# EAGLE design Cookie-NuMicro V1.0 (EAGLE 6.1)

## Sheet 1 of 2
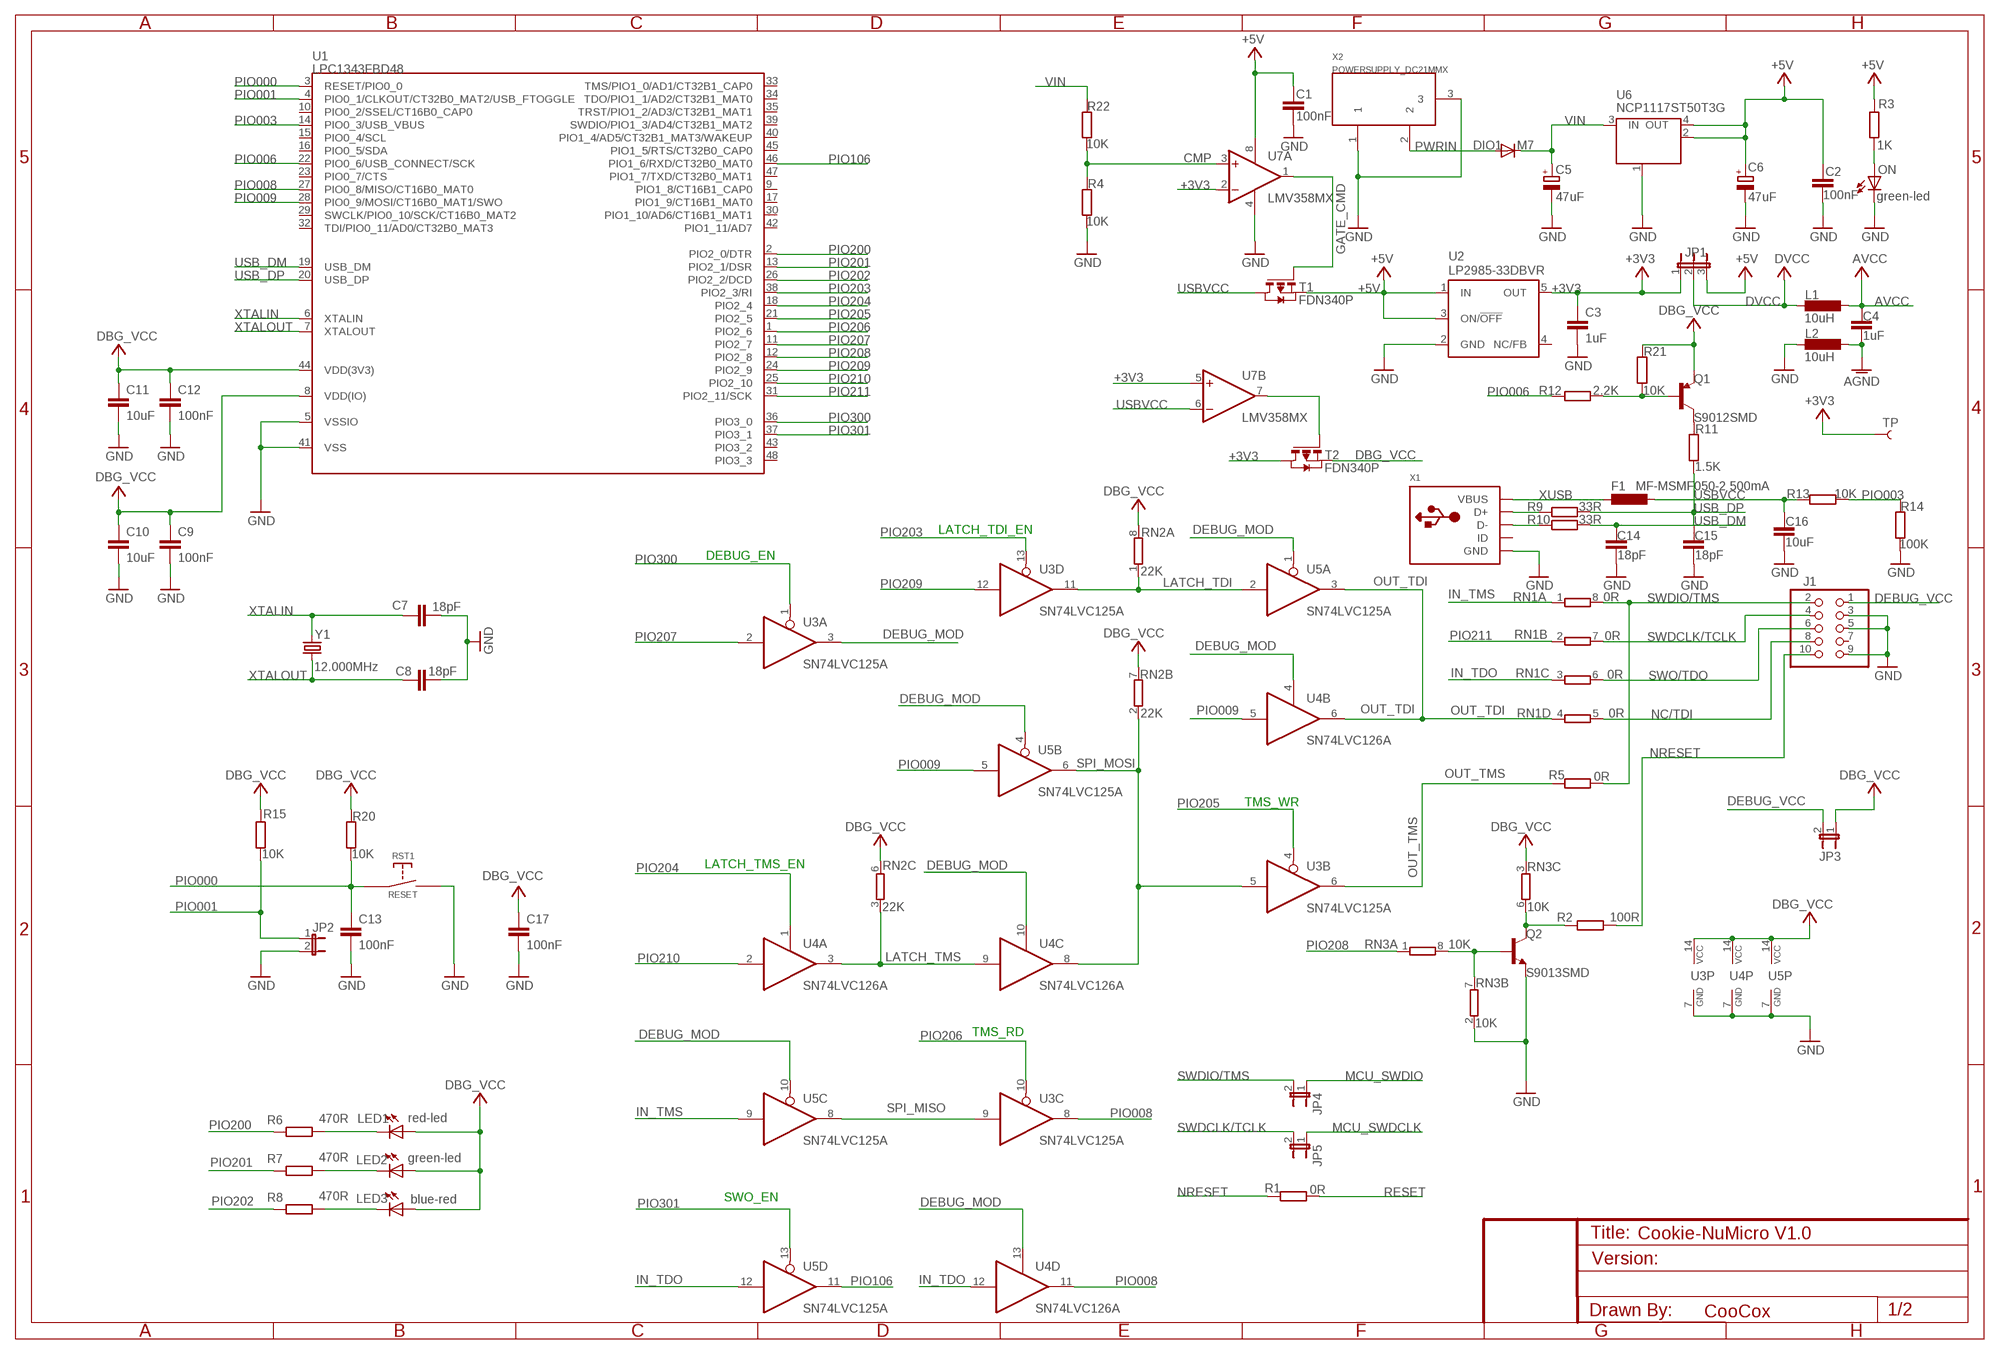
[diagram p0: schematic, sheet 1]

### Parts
C1  100nF  C-EUC0603  [C0603]
C2  100nF  C-EUC0603  [C0603]
C3  1uF  C-EUC0603  [C0603]
C4  1uF  C-EUC0603  [C0603@1]
C5  47uF  CPOL-EUD  [PANASONIC_D]
C6  47uF  CPOL-EUD  [PANASONIC_D]
C7  18pF  C-EUC0603  [C0603@1]
C8  18pF  C-EUC0603  [C0603@1]
C9  100nF  C-EUC0603  [C0603@1]
C10  10uF  C-EUC0805  [C0805]
C11  10uF  C-EUC0805  [C0805]
C12  100nF  C-EUC0603  [C0603@1]
C13  100nF  C-EUC0603  [C0603@1]
C14  18pF  C-EUC0603  [C0603@1]
C15  18pF  C-EUC0603  [C0603]
C16  10uF  C-EUC0805  [C0805]
C17  100nF  C-EUC0603  [C0603@1]
DIO1  M7  DIODE-SMB  [SMB]
F1  MF-MSMF050-2 500mA  L-EUL1812  [L1812]
J1  PINHD-2X5  [2X05]
JP1  JP2E  [JP2]
JP2  JP1E  [JP1]
JP3  JP1E  [JP1]
JP4  JP1E  [JP1]
JP5  JP1E  [JP1]
L1  10uH  L-EUL3216C  [L3216C]
L2  10uH  L-EUL3216C  [L3216C]
LED1  red-led  LEDCHIP-LED0805  [CHIP-LED0805]
LED2  green-led  LEDCHIP-LED0805  [CHIP-LED0805]
LED3  blue-red  LEDCHIP-LED0805  [CHIP-LED0805]
ON  green-led  LEDCHIP-LED0805  [CHIP-LED0805]
Q1  S9012SMD  TRANSISTOR_PNPSMD  [SOT23-3]
Q2  S9013SMD  TRANSISTOR_NPNSOT23  [SOT23]
R1  0R  R-EU_R0603  [R0603]
R2  100R  R-EU_R0603  [R0603]
R3  1K  R-EU_R0603  [R0603]
R4  10K  R-EU_R0603  [R0603]
R5  0R  R-EU_R0603  [R0603]
R6  470R  R-EU_R0603  [R0603]
R7  470R  R-EU_R0603  [R0603]
R8  470R  R-EU_R0603  [R0603]
R9  33R  R-EU_R0603  [R0603]
R10  33R  R-EU_R0603  [R0603]
R11  1.5K  R-EU_R0603  [R0603]
R12  2.2K  R-EU_R0603  [R0603]
R13  10K  R-EU_R0603  [R0603]
R14  100K  R-EU_R0603  [R0603]
R15  10K  R-EU_R0603  [R0603]
R20  10K  R-EU_R0603  [R0603]
R21  10K  R-EU_R0603  [R0603]
R22  10K  R-EU_R0603  [R0603]
RN1  0R  4R-N0603-ARV  [0603-ARV]
RN2  22K  4R-N0603-ARV  [0603-ARV]
RN3  10K  4R-N0603-ARV  [0603-ARV]
RST1  RESET  SWITCH  [TACTILE-SWITCH-1101NE]
T1  FDN340P  PMOSSOT23  [SOT-23]
T2  FDN340P  PMOSSOT23  [SOT-23]
TP  TEST-POINT3X5  [PAD.03X.05]
U1  LPC1343FBD48  [LQFP48-7X7]
U2  LP2985-33DBVR  LP2985-XXDBVR33  [SOT23-DBV]
U3  SN74LVC125A  74LVC125A  [TSSOP14]
U4  SN74LVC126A  74LVC126A  [TSSOP14]
U5  SN74LVC125A  74LVC125A  [TSSOP14]
U6  NCP1117ST50T3G  MC33269ST-3.3T3  [SOT223]
U7  LMV358MX  [SO08]
X1  USBMINIB  [USB-MINIB]
X2  POWERSUPPLY_DC21MMX  [POWERSUPPLY_DC-21MM]
Y1  12.000MHz  MC-405  [MC-405]

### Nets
+3V3: C3.1 JP1.1 T2.1(D) TP.P$1 U2.5(OUT) U7.2(A:-IN) U7.5(B:+IN) ; also sheet 2
+5V [usbvcc]: C1.1 C2.1 C6.+ JP1.3 R3.1 T1.2(S) U2.1(IN) U2.3(ON/!OFF) U6.2(OUT) U6.4(OUT) U7.8(P:V+) ; also sheet 2
AGND: C4.2 L2.2 ; also sheet 2
AVCC: C4.1 L1.2 ; also sheet 2
CMP: R4.2 R22.1 U7.3(A:+IN)
DBG_VCC [gnd]: C9.1 C10.1 C11.1 C12.1 C17.1 JP3.1 LED1.A LED2.A LED3.A Q1.2(E) R15.1 R20.2 R21.2 RN2.6 RN2.7 RN2.8 RN3.3 T2.2(S) U1.8(VDD(IO)) U1.44(VDD(3V3)) U3.14(P:VCC) U4.14(P:VCC) U5.14(P:VCC)
DEBUG_MOD: U3.3(A:O) U4.4(B:OE) U4.10(C:OE) U4.13(D:OE) U5.1(A:OE) U5.4(B:OE) U5.10(C:OE)
DEBUG_VCC: J1.1 JP3.2
DVCC: JP1.2 L1.1 ; also sheet 2
GATE_CMD: T1.3(G) U7.1(A:OUT)
GND [gnd]: C1.2 C2.2 C3.2 C5.- C6.- C7.1 C8.2 C9.2 C10.2 C11.2 C12.2 C13.2 C14.1 C15.1 C16.1 C17.2 J1.3 J1.5 J1.9 JP2.2 L2.1 ON.C Q2.2(E) R4.1 R14.1 RN3.2 RST1.P$2 U1.5(VSSIO) U1.41(VSS) U2.2(GND) U3.7(P:GND) U4.7(P:GND) U5.7(P:GND) U6.1(GND/ADJ) U7.4(P:V-) X1.GND X2.1 X2.3 ; also sheet 2
IN_TDO: RN1.3 U4.12(D:I) U5.12(D:I)
IN_TMS: RN1.1 U5.9(C:I)
LATCH_TDI: RN2.1 U3.11(D:O) U5.2(A:I)
LATCH_TMS: RN2.3 U4.3(A:O) U4.9(C:I)
MCU_SWDCLK: JP5.1 ; also sheet 2
MCU_SWDIO: JP4.1 ; also sheet 2
N$1: ON.A R3.2
N$7: T2.3(G) U7.7(B:OUT)
N$13: R9.2 X1.D+
N$14: Q1.3(C) R11.2
N$15: R10.2 X1.D-
N$16: Q1.1(B) R12.2 R21.1
N$17: LED3.C R8.2
N$19: LED2.C R7.2
N$32: LED1.C R6.2
N$33: Q2.3(C) R2.1 RN3.6
N$41: Q2.1(B) RN3.7 RN3.8
NC/TDI: J1.8 RN1.5
NRESET: J1.10 R1.2 R2.2
OUT_TDI: RN1.4 U4.6(B:O) U5.3(A:O)
OUT_TMS: R5.2 U3.6(B:O)
PIO000: C13.1 R20.1 RST1.P$1 U1.3(RESET/PIO0_0)
PIO001: JP2.1 R15.2 U1.4(PIO0_1/CLKOUT/CT32B0_MAT2/USB_FTOGGLE)
PIO003: R13.2 R14.2 U1.14(PIO0_3/USB_VBUS)
PIO006: R12.1 U1.22(PIO0_6/USB_CONNECT/SCK)
PIO008: U1.27(PIO0_8/MISO/CT16B0_MAT0) U3.8(C:O) U4.11(D:O)
PIO009: U1.28(PIO0_9/MOSI/CT16B0_MAT1/SWO) U4.5(B:I) U5.5(B:I)
PIO106: U1.46(PIO1_6/RXD/CT32B0_MAT0) U5.11(D:O)
PIO200: R6.1 U1.2(PIO2_0/DTR)
PIO201: R7.1 U1.13(PIO2_1/DSR)
PIO202: R8.1 U1.26(PIO2_2/DCD)
PIO203: U1.38(PIO2_3/RI) U3.13(D:OE)
PIO204: U1.18(PIO2_4) U4.1(A:OE)
PIO205: U1.21(PIO2_5) U3.4(B:OE)
PIO206: U1.1(PIO2_6) U3.10(C:OE)
PIO207: U1.11(PIO2_7) U3.2(A:I)
PIO208: RN3.1 U1.12(PIO2_8)
PIO209: U1.24(PIO2_9) U3.12(D:I)
PIO210: U1.25(PIO2_10) U4.2(A:I)
PIO211: RN1.2 U1.31(PIO2_11/SCK)
PIO300: U1.36(PIO3_0) U3.1(A:OE)
PIO301: U1.37(PIO3_1) U5.13(D:OE)
PWRIN [power]: DIO1.A X2.2
RESET: R1.1 ; also sheet 2
SPI_MISO: U3.9(C:I) U5.8(C:O)
SPI_MOSI: RN2.2 U3.5(B:I) U4.8(C:O) U5.6(B:O)
SWDCLK/TCLK: J1.4 JP5.2 RN1.7
SWDIO/TMS: J1.2 JP4.2 R5.1 RN1.8
SWO/TDO: J1.6 RN1.6
USB_DM: C14.2 R10.1 U1.19(USB_DM)
USB_DP: C15.2 R9.1 R11.1 U1.20(USB_DP)
USBVCC [usbvcc]: C16.2 F1.1 R13.1 T1.1(D) U7.6(B:-IN)
VIN [power]: C5.+ DIO1.C R22.2 U6.3(IN) ; also sheet 2
XTALIN: C7.2 U1.6(XTALIN) Y1.2
XTALOUT: C8.1 U1.7(XTALOUT) Y1.1
XUSB: F1.2 X1.VBUS
Unconnected: J1.7 RN2.4 RN2.5 RN3.4 RN3.5 U1.9(PIO1_8/CT16B1_CAP0) U1.10(PIO0_2/SSEL/CT16B0_CAP0) U1.15(PIO0_4/SCL) U1.16(PIO0_5/SDA) U1.17(PIO1_9/CT16B1_MAT0) U1.23(PIO0_7/CTS) U1.29(SWCLK/PIO0_10/SCK/CT16B0_MAT2) U1.30(PIO1_10/AD6/CT16B1_MAT1) U1.32(TDI/PIO0_11/AD0/CT32B0_MAT3) U1.33(TMS/PIO1_0/AD1/CT32B1_CAP0) U1.34(TDO/PIO1_1/AD2/CT32B1_MAT0) U1.35(TRST/PIO1_2/AD3/CT32B1_MAT1) U1.39(SWDIO/PIO1_3/AD4/CT32B1_MAT2) U1.40(PIO1_4/AD5/CT32B1_MAT3/WAKEUP) U1.42(PIO1_11/AD7) U1.43(PIO3_2) U1.45(PIO1_5/RTS/CT32B0_CAP0) U1.47(PIO1_7/TXD/CT32B0_MAT1) U1.48(PIO3_3) U2.4(NC/FB) X1.ID

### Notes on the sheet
- LATCH_TDI_EN
- DEBUG_EN
- TMS_WR
- LATCH_TMS_EN
- TMS_RD
- SWO_EN
- CooCox

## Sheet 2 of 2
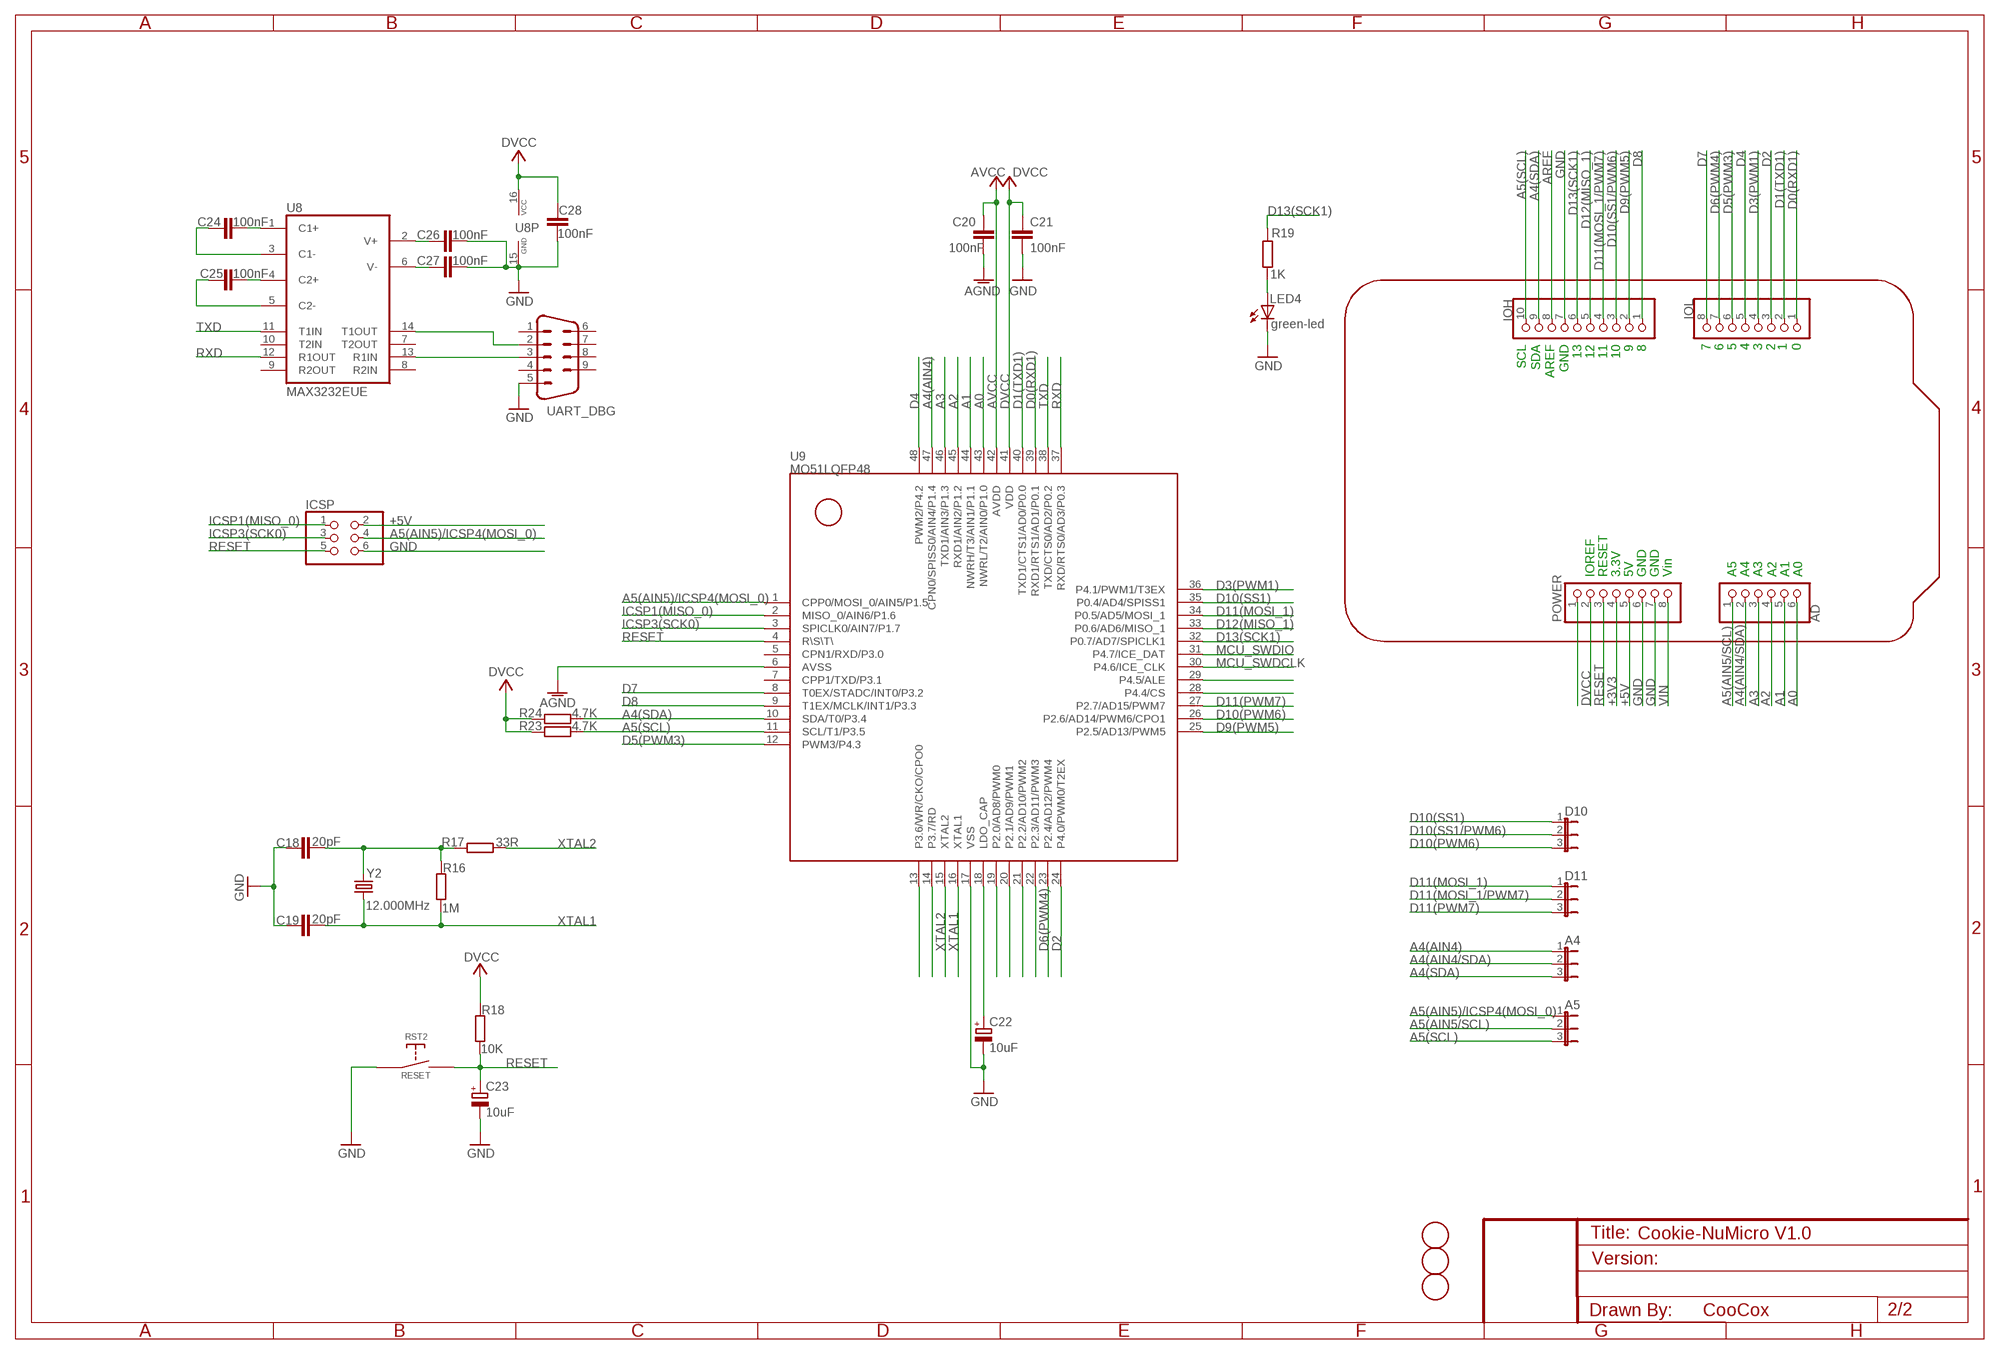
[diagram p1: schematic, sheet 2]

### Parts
A4  JP2E  [JP2]
A5  JP2E  [JP2]
AD  PINHD-1X6  [1X06]
C18  20pF  C-EUC0603  [C0603@1]
C19  20pF  C-EUC0603  [C0603@1]
C20  100nF  C-EUC0603  [C0603@1]
C21  100nF  C-EUC0603  [C0603@1]
C22  10uF  CPOL-EUSMCB  [SMC_B]
C23  10uF  CPOL-EUSMCB  [SMC_B]
C24  100nF  C-EUC0603  [C0603@1]
C25  100nF  C-EUC0603  [C0603@1]
C26  100nF  C-EUC0603  [C0603@1]
C27  100nF  C-EUC0603  [C0603@1]
C28  100nF  C-EUC0603  [C0603@1]
D10  JP2E  [JP2]
D11  JP2E  [JP2]
FD1  FIDUCIALMOUNT  [FIDUCIA-MOUNT]
FD2  FIDUCIALMOUNT  [FIDUCIA-MOUNT]
FD3  FIDUCIALMOUNT  [FIDUCIA-MOUNT]
ICSP  PINHD-2X3  [2X03]
IOH  PINHD-1X10_ARD  [1X10]
IOL  PINHD-1X8  [1X08]
LED4  green-led  LEDCHIP-LED0805  [CHIP-LED0805]
POWER  PINHD-1X8  [1X08]
R16  1M  R-EU_R0603  [R0603]
R17  33R  R-EU_R0603  [R0603]
R18  10K  R-EU_R0603  [R0603]
R19  1K  R-EU_R0603  [R0603]
R23  4.7K  R-EU_R0603  [R0603]
R24  4.7K  R-EU_R0603  [R0603]
RST2  RESET  SWITCH  [TACTILE-SWITCH-1101NE]
U8  MAX3232EUE  [TSSOP16]
U9  MO51LQFP48  [LQFP48]
UART_DBG  M09S_OBVERSE  [M09S_OBV]
Y2  12.000MHz  MC-405  [MC-405]

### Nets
+3V3: POWER.4 ; also sheet 1
+5V [usbvcc]: ICSP.2 POWER.5 ; also sheet 1
A0: AD.6 U9.43(NWRL/T2/AIN0/P1.0)
A1: AD.5 U9.44(NWRH/T3/AIN1/P1.1)
A2: AD.4 U9.45(RXD1/AIN2/P1.2)
A3: AD.3 U9.46(TXD1/AIN3/P1.3)
A4(AIN4): A4.1 U9.47(CPN0/SPISS0/AIN4/P1.4)
A4(AIN4/SDA): A4.2 AD.2
A4(SDA): A4.3 IOH.9 R24.1 U9.10(SDA/T0/P3.4)
A5(AIN5)/ICSP4(MOSI_0): A5.1 ICSP.4 U9.1(CPP0/MOSI_0/AIN5/P1.5)
A5(AIN5/SCL): A5.2 AD.1
A5(SCL): A5.3 IOH.10 R23.1 U9.11(SCL/T1/P3.5)
AGND: C20.2 U9.6(AVSS) ; also sheet 1
AREF: IOH.8
AVCC: C20.1 U9.42(AVDD) ; also sheet 1
D0(RXD1): IOL.1 U9.39(RXD1/RTS1/AD1/P0.1)
D1(TXD1): IOL.2 U9.40(TXD1/CTS1/AD0/P0.0)
D2: IOL.3 U9.24(P4.0/PWM0/T2EX)
D3(PWM1): IOL.4 U9.36(P4.1/PWM1/T3EX)
D4: IOL.5 U9.48(PWM2/P4.2)
D5(PWM3): IOL.6 U9.12(PWM3/P4.3)
D6(PWM4): IOL.7 U9.23(P2.4/AD12/PWM4)
D7: IOL.8 U9.8(T0EX/STADC/INT0/P3.2)
D8: IOH.1 U9.9(T1EX/MCLK/INT1/P3.3)
D9(PWM5): IOH.2 U9.25(P2.5/AD13/PWM5)
D10(PWM6): D10.3 U9.26(P2.6/AD14/PWM6/CPO1)
D10(SS1): D10.1 U9.35(P0.4/AD4/SPISS1)
D10(SS1/PWM6): D10.2 IOH.3
D11(MOSI_1): D11.1 U9.34(P0.5/AD5/MOSI_1)
D11(MOSI_1/PWM7): D11.2 IOH.4
D11(PWM7): D11.3 U9.27(P2.7/AD15/PWM7)
D12(MISO_1): IOH.5 U9.33(P0.6/AD6/MISO_1)
D13(SCK1): IOH.6 R19.1 U9.32(P0.7/AD7/SPICLK1)
DVCC: C21.1 C28.1 POWER.2 R18.2 R23.2 R24.2 U8.16(VCC) U9.41(VDD) ; also sheet 1
GND [gnd]: C18.1 C19.1 C21.2 C22.- C23.- C26.2 C27.2 C28.2 ICSP.6 IOH.7 LED4.C POWER.6 POWER.7 RST2.P$1 U8.15(GND) U9.17(VSS) UART_DBG.5 ; also sheet 1
ICSP1(MISO_0): ICSP.1 U9.2(MISO_0/AIN6/P1.6)
ICSP3(SCK0): ICSP.3 U9.3(SPICLK0/AIN7/P1.7)
MCU_SWDCLK: U9.30(P4.6/ICE_CLK) ; also sheet 1
MCU_SWDIO: U9.31(P4.7/ICE_DAT) ; also sheet 1
N$2: LED4.A R19.2
N$3: C24.2 U8.1(C1+)
N$4: C24.1 U8.3(C1-)
N$5: C25.2 U8.4(C2+)
N$6: C25.1 U8.5(C2-)
N$8: U8.14(T1OUT) UART_DBG.2
N$9: U9.29(P4.5/ALE)
N$10: U9.28(P4.4/CS)
N$11: C26.1 U8.2(V+)
N$12: C27.1 U8.6(V-)
N$36: POWER.1
N$38: U9.13(P3.6/WR/CKO/CPO0)
N$39: U9.14(P3.7/RD)
N$40: C18.2 R16.2 R17.2 Y2.2
N$42: U8.13(R1IN) UART_DBG.3
N$43: C22.+ U9.18(LDO_CAP)
N$44: U9.19(P2.0/AD8/PWM0)
N$45: U9.20(P2.1/AD9/PWM1)
N$46: U9.21(P2.2/AD10/PWM2)
N$47: U9.22(P2.3/AD11/PWM3)
RESET: C23.+ ICSP.5 POWER.3 R18.1 RST2.P$2 U9.4(R\S\T\) ; also sheet 1
RXD: U8.12(R1OUT) U9.37(RXD/RTS0/AD3/P0.3)
TXD: U8.11(T1IN) U9.38(TXD/CTS0/AD2/P0.2)
VIN [power]: POWER.8 ; also sheet 1
XTAL1: C19.2 R16.1 U9.16(XTAL1) Y2.1
XTAL2: R17.1 U9.15(XTAL2)
Unconnected: U8.7(T2OUT) U8.8(R2IN) U8.9(R2OUT) U8.10(T2IN) U9.5(CPN1/RXD/P3.0) U9.7(CPP1/TXD/P3.1) UART_DBG.1 UART_DBG.4 UART_DBG.6 UART_DBG.7 UART_DBG.8 UART_DBG.9

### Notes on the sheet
- SCL | SDA | AREF | GND | 13 | 12 | 11 | 10 | 9 | 8 | 7 | 6 | 5 | 4 | 3 | 2 | 1 | 0
- IOREF | RESET | 3.3V | 5V | GND | GND | Vin | A5 | A4 | A3 | A2 | A1 | A0
- CooCox

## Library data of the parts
A4 A5 D10 D11 JP1 = jumper:JP2E: JUMPER
AD = SmartPrj:PINHD-1X6: PIN HEADER
C1-C3 C15 C16 = resistor:C-EU: CAPACITOR, European symbol
C4 C7-C14 C17-C21 C24-C28 = rcl:C-EU: CAPACITOR, European symbol
C5 C6 C22 C23 = rcl:CPOL-EU: POLARIZED CAPACITOR, European symbol
DIO1 = diode:DIODE-: DIODE
F1 L1 L2 = rcl:L-EU: INDUCTOR, European symbol
FD1-FD3 = SmartPrj:FIDUCIALMOUNT
ICSP = pinhead:PINHD-2X3: PIN HEADER
IOH = SmartPrj:PINHD-1X10_ARD: PIN HEADER
IOL POWER = SmartPrj:PINHD-1X8: PIN HEADER
J1 = pinhead:PINHD-2X5: PIN HEADER
JP2-JP5 = jumper:JP1E: JUMPER
LED1-LED4 ON = led:LED: LED
Q1 = SparkFunEagle-100301:TRANSISTOR_PNP
Q2 = SparkFunEagle-100301:TRANSISTOR_NPN: Transistor NPN BJT configuration in SOT23 package. MMBT2222 is the common NPN we use. Double check BCE configuration again layout.
R1 R3-R12 R15-R24 = rcl:R-EU_: RESISTOR, European symbol
R2 R13 R14 = resistor:R-EU_: RESISTOR, European symbol
RN1-RN3 = resistor-dil:4R-N: Array Chip Resistor Source: RS Component / Phycomp; OC_FARNELL: unknown; OC_NEWARK: unknown
RST1 RST2 = SWITCH1:SWITCH
T1 T2 = zetex:PMOSSOT23: MOS FET
TP = SparkFunEagle-100301:TEST-POINT
U1 = lpc1xxx-v6:LPC1343FBD48: LPC1343 72 MHz 32-bit ARM Cortex-M3 based microcontroller featuring a high level of integration and low power consumption. 32 kB Flash, 8 kB SRAM, USB Device MarcVl - Datasheet available on www.nxp.com
U2 = SmartPrj:LP2985-XXDBVR: ULTRALOW-POWER 50-mA LOW-DROPOUT LINEAR REGULATORS 50-mA Low-Dropout Regulator Source: http://focus.ti.com/lit/ds/symlink/tps77001.pdf
U3 U5 = 74xx-eu:74*125: Quad bus BUFFER, 3-state
U4 = 74xx-eu:74*126: Quad bus BUFFER, 3-state
U6 = linear:MC33269ST*: Adjustable Output Low Dropout Voltage Regulator 800 mA Source: http://www.onsemi.com/pub/Collateral/MC33269-D.PDF
U7 = linear:LMV358?*: Dual General Purpose, Low Voltage, Rail-to-Rail Output Operational Amplifiers Source: http://www.national.com/mpf/LM/LMV321.html http://www.national.com/dt/lmv_qual.pdf
U8 = maxim:MAX3232*: True RS-232 Transceivers 3.0V to 5.5V, Low-Power up to 1Mbps, Using Four 0.1µF External Capacitors Source: http://pdfserv.maxim-ic.com/en/ds/MAX3222-MAX3241.pdf; MF: MAXIM; MPN: MAX3232EUE+; OC_FARNELL: 1379769; OC_NEWARK: 68K4632
U9 = NuMicro:MO51
UART_DBG = con-subd:M09: SUB-D
X1 = adafruit:USB: USB Connectors USBMINIB - Surface Mount Female Mini-B USB Connector 4UConnector: 06564 By microbuilder.eu Thru-hole RA Female Mini-B USB Connector 4UConnector: 18732 By ladyada.net
X2 = SmartPrj:POWERSUPPLY_DC21MM
Y1 Y2 = untitled:MC-405: kHz RANGE CRYSTAL UNIT SMD; OC_FARNELL: unknown; OC_NEWARK: unknown

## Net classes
1 power: width 0.61 mm, drill 0.61 mm, clearance 0.254 mm
2 gnd: width 0.305 mm, drill 0.559 mm, clearance 0.254 mm
3 usbvcc: width 0.508 mm, drill 0.61 mm, clearance 0.254 mm

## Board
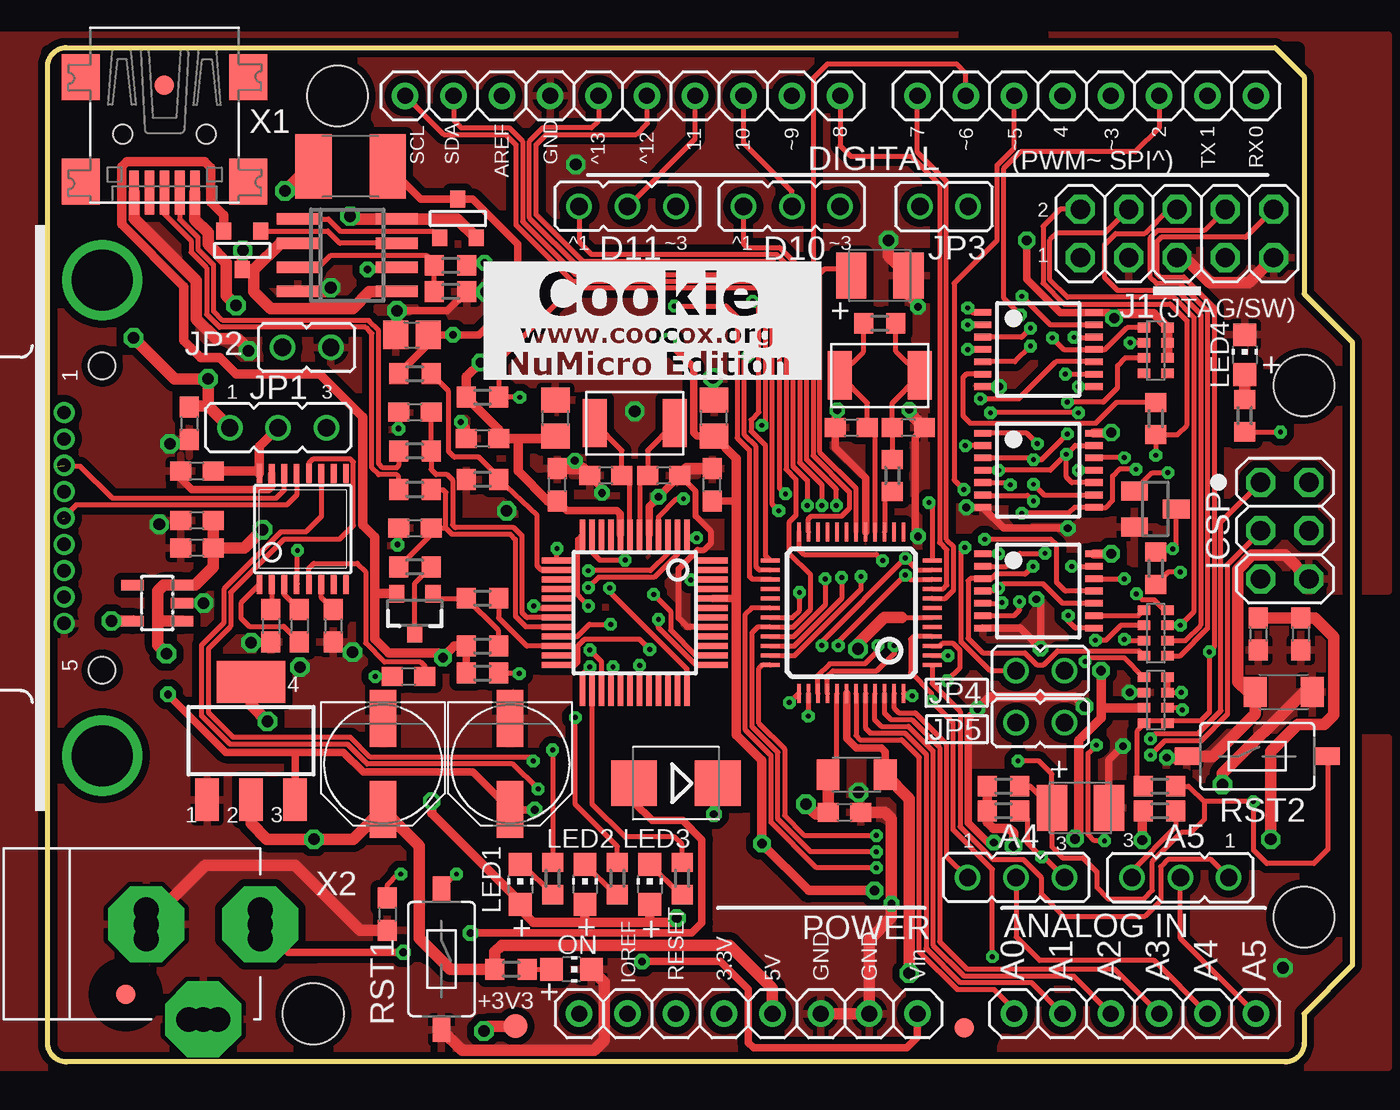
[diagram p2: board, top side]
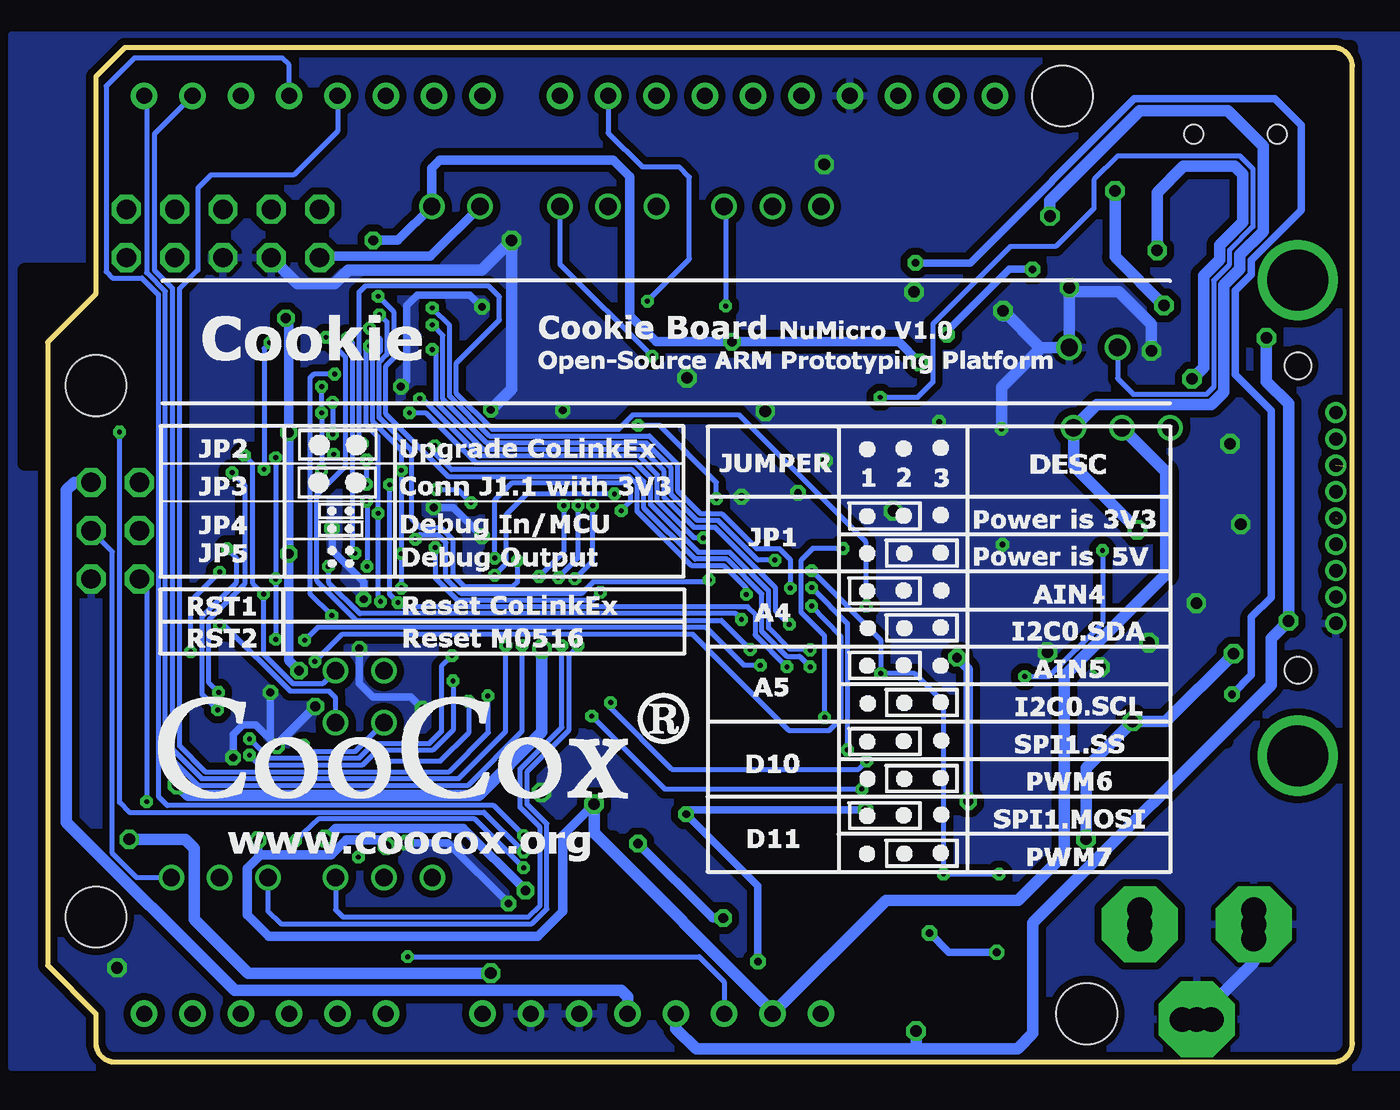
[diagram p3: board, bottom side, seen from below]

Size 68.58 x 53.34 mm. Coordinates in mm from the lower left corner, seen from the top.
Outline: 64.52,53.34 66.04,51.82 66.04,40.39 68.58,37.85 68.58,5.08 66.04,2.54 66.04,1 arc-90 65.04,0 1,0 arc-90 0,1 0,52.34 arc-90 1,53.34 64.52,53.34
Copper layers (1*16): Top 0.035mm / dielectric 1.5mm / Bottom 0.035mm
Design rules: minimum track width 6mil, minimum drill 6mil, track to track 4mil, track to pad 4mil, pad to pad 4mil, via to via 4mil, smd to smd 0mil, copper to edge 10mil, drill to drill 6mil, minimum pad ring 8mil, minimum via ring 8mil, stop-mask expansion 0mil, vias tented up to drill 100mil, thermal gap 10mil
Holes 3.2 mm at 66.04,35.56 66.04,7.62 15.24,50.8 13.97,2.54
tRestrict: area 3.1,2.5 to 5.1,4.6; area 47.2,0.8 to 49.2,2.8; area 5.1,50.3 to 7.2,52.4; area 9.7,43.9 to 10.7,44.9; area 5.3,37.9 to 6,41.4; area 4.9,38.4 to 5.3,40.5; area 4.4,38.6 to 5,39.9; area 5.9,37.3 to 6.5,40.9; area 6.2,36.6 to 7.2,37.6; area 0.3,42.4 to 3.6,45.1; area 0,46.9 to 14.9,53.1; area 14.9,45.1 to 16.8,49.2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
bRestrict: area 2.7,20.5 to 3.1,20.9; area 2.7,36.5 to 3.1,36.9; area 45.1,29.6 to 46.6,30.7; area 48.3,32.8 to 49.4,33.8; area 48.2,30.6 to 49,31.3; area 54.3,22.8 to 55.7,24.3; area 57.2,22.5 to 59.3,24.5; area 44.6,19.3 to 47.3,22.3; area 44.1,13 to 45.1,14.7; area 61.6,8 to 62.5,9.1; area 62.5,10 to 64.7,11.3; area 65.9,8.6 to 68.1,11.9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

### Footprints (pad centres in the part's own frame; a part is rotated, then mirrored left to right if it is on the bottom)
JP2 = drill 0.914 long: 1 -2.54,0; 2 0,0; 3 2.54,0
1X06 = drill 0.85 pad 1.422 long: 1 -6.35,0; 2 -3.81,0; 3 -1.27,0; 4 1.27,0; 5 3.81,0; 6 6.35,0
C0603 = smd 1.1 x 1: 1 -0.85,0; 2 0.85,0
PANASONIC_D = smd 3 x 1.4: + 2.4,0; - -2.4,0
C0805 = smd 1.3 x 1.5: 1 -0.95,0; 2 0.95,0
C0805' = smd 1.3 x 1.5: 1 -0.85,0; 2 0.85,0
SMC_B = smd 1.6 x 2.4: + -1.5,0; - 1.5,0
SMB = smd 2.4 x 2.4: A 2.2,0; C -2.2,0
L1812 = smd 1.9 x 3.4: 1 -1.95,0; 2 1.95,0
FIDUCIA-MOUNT = smd 1.016 x 1.016: P$1 0,0
2X03 = drill 1.016 octagon: 1 -2.54,-1.27; 2 -2.54,1.27; 3 0,-1.27; 4 0,1.27; 5 2.54,-1.27; 6 2.54,1.27
1X10 = drill 0.85 pad 1.422 long: 1 -11.43,0; 2 -8.89,0; 3 -6.35,0; 4 -3.81,0; 5 -1.27,0; 6 1.27,0; 7 3.81,0; 8 6.35,0; 9 8.89,0; 10 11.43,0
1X08 = drill 0.85 pad 1.422 long: 1 -8.89,0; 2 -6.35,0; 3 -3.81,0; 4 -1.27,0; 5 1.27,0; 6 3.81,0; 7 6.35,0; 8 8.89,0
2X05 = drill 1.016 octagon: 1 -5.08,-1.27; 2 -5.08,1.27; 3 -2.54,-1.27; 4 -2.54,1.27; 5 0,-1.27; 6 0,1.27; 7 2.54,-1.27; 8 2.54,1.27; 9 5.08,-1.27; 10 5.08,1.27
JP1 = drill 0.914 long: 1 0,-1.27; 2 0,1.27
L3216C = smd 1.2 x 1.6: 1 -1.5,0; 2 1.5,0
CHIP-LED0805 = smd 1.2 x 1.2: A 0,-1.05; C 0,1.05
SOT23-3 = smd 0.8 x 0.9: 1 -0.95,-1; 2 0.95,-1; 3 0,1.1
SOT23 = smd 1 x 1.4: 1 -0.95,-1.1; 2 0.95,-1.1; 3 0,1.1
R0603 = smd 1 x 1.1: 1 -0.85,0; 2 0.85,0
0603-ARV = smd 0.5 x 0.65: 1 -1.2,-0.625; 2 -0.4,-0.625; 3 0.4,-0.625; 4 1.2,-0.625; 5 1.2,0.625; 6 0.4,0.625; 7 -0.4,0.625; 8 -1.2,0.625
TACTILE-SWITCH-1101NE = smd 1.27 x 0.914: P$1 -3.708,0; P$2 3.708,0
SOT-23 = smd 0.787 x 0.889: 1 0.025,-1.016; 2 -0.94,1.016; 3 0.991,1.016
PAD.03X.05 = smd 1.27 x 1.27: P$1 0,0
LQFP48-7X7 = smd 0.3 x 1.6: 1 -2.75,-4.1; 2 -2.25,-4.1; 3 -1.75,-4.1; 4 -1.25,-4.1; 5 -0.75,-4.1; 6 -0.25,-4.1; 7 0.25,-4.1; 8 0.75,-4.1; 9 1.25,-4.1; 10 1.75,-4.1; 11 2.25,-4.1; 12 2.75,-4.1; 25 2.75,4.1; 26 2.25,4.1; 27 1.75,4.1; 28 1.25,4.1; 29 0.75,4.1; 30 0.25,4.1; 31 -0.25,4.1; 32 -0.75,4.1; 33 -1.25,4.1; 34 -1.75,4.1; 35 -2.25,4.1; 36 -2.75,4.1 | smd 1.6 x 0.3: 13 4.1,-2.75; 14 4.1,-2.25; 15 4.1,-1.75; 16 4.1,-1.25; 17 4.1,-0.75; 18 4.1,-0.25; 19 4.1,0.25; 20 4.1,0.75; 21 4.1,1.25; 22 4.1,1.75; 23 4.1,2.25; 24 4.1,2.75; 37 -4.1,2.75; 38 -4.1,2.25; 39 -4.1,1.75; 40 -4.1,1.25; 41 -4.1,0.75; 42 -4.1,0.25; 43 -4.1,-0.25; 44 -4.1,-0.75; 45 -4.1,-1.25; 46 -4.1,-1.75; 47 -4.1,-2.25; 48 -4.1,-2.75
SOT23-DBV = smd 0.55 x 1.2: 1 -0.95,-1.3; 2 0,-1.3; 3 0.95,-1.3; 4 0.95,1.3; 5 -0.95,1.3
TSSOP14 = smd 0.35 x 0.9: 1 -1.95,-2.925; 2 -1.3,-2.925; 3 -0.65,-2.925; 4 0,-2.925; 5 0.65,-2.925; 6 1.3,-2.925; 7 1.95,-2.925; 8 1.95,2.925; 9 1.3,2.925; 10 0.65,2.925; 11 0,2.925; 12 -0.65,2.925; 13 -1.3,2.925; 14 -1.95,2.925
SOT223 = smd 1.219 x 2.235: 1 -2.311,-3.099; 2 0,-3.099; 3 2.311,-3.099 | smd 3.6 x 2.2: 4 0,3.099
SO08 = smd 0.6 x 2.2: 1 -1.905,-2.6; 2 -0.635,-2.6; 3 0.635,-2.6; 4 1.905,-2.6; 5 1.905,2.6; 6 0.635,2.6; 7 -0.635,2.6; 8 -1.905,2.6
TSSOP16 = smd 0.305 x 0.991: 1 -2.275,-2.918; 2 -1.625,-2.918; 3 -0.975,-2.918; 4 -0.325,-2.918; 5 0.325,-2.918; 6 0.975,-2.918; 7 1.625,-2.918; 8 2.275,-2.918; 9 2.275,2.918; 10 1.625,2.918; 11 0.975,2.918; 12 0.325,2.918; 13 -0.325,2.918; 14 -0.975,2.918; 15 -1.625,2.918; 16 -2.275,2.918
LQFP48 = smd 0.2 x 1: 1 -2.75,-4.25; 2 -2.25,-4.25; 3 -1.75,-4.25; 4 -1.25,-4.25; 5 -0.75,-4.25; 6 -0.25,-4.25; 7 0.25,-4.25; 8 0.75,-4.25; 9 1.25,-4.25; 10 1.75,-4.25; 11 2.25,-4.25; 12 2.75,-4.25; 25 2.75,4.25; 26 2.25,4.25; 27 1.75,4.25; 28 1.25,4.25; 29 0.75,4.25; 30 0.25,4.25; 31 -0.25,4.25; 32 -0.75,4.25; 33 -1.25,4.25; 34 -1.75,4.25; 35 -2.25,4.25; 36 -2.75,4.25 | smd 1 x 0.2: 13 4.25,-2.75; 14 4.25,-2.25; 15 4.25,-1.75; 16 4.25,-1.25; 17 4.25,-0.75; 18 4.25,-0.25; 19 4.25,0.25; 20 4.25,0.75; 21 4.25,1.25; 22 4.25,1.75; 23 4.25,2.25; 24 4.25,2.75; 37 -4.25,2.75; 38 -4.25,2.25; 39 -4.25,1.75; 40 -4.25,1.25; 41 -4.25,0.75; 42 -4.25,0.25; 43 -4.25,-0.25; 44 -4.25,-0.75; 45 -4.25,-1.25; 46 -4.25,-1.75; 47 -4.25,-2.25; 48 -4.25,-2.75
M09S_OBV = drill 0.7: 1 5.34,2; 2 2.57,2; 3 -0.2,2; 4 -2.97,2; 5 -5.74,2; 6 3.955,2; 7 1.185,2; 8 -1.585,2; 9 -4.355,2 | drill 3.2: P$1 -12.7,0; P$2 12.3,0 | hole 1.4: -8.2,0; 7.8,0
USB-MINIB = smd 0.5 x 2.308: D+ 0,4.064; D- -0.8,4.064; GND 1.6,4.064; ID 0.8,4.064; VBUS -1.6,4.064 | smd 2 x 2.4: GND1 -4.4,-2; GND2 -4.4,3.5; GND3 4.4,3.5; GND4 4.4,-2 | hole 1: -2.2,1; 2.2,1
POWERSUPPLY_DC-21MM = drill 1.3 pad 4 octagon: 1 -5.08,-3.353; 2 -0.076,-6.35; 3 -0.076,-0.356 | drill 1.3: 4 -5.08,-4.115; 5 -5.08,-2.591; 6 -0.838,-0.356; 7 0.686,-0.356; 8 -0.838,-6.35; 9 0.686,-6.35
MC-405 = smd 1.27 x 2.54: 1 -2.108,0.013; 2 2.108,0.012

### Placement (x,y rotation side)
A4  50.9,9.7 0 top
A5  59.54,9.7 180 top
AD  57.15,2.54 180 top
C1  7.85,27.03 180 top
C2  7.85,28.47 180 top
C3  7.44,33.58 270 top
C4  1uF  [C0603]  63.63,22.5 270 top
C5  24.31,15.67 270 top
C6  17.63,15.67 270 top
C7  18pF  [C0603]  32.38,30.84 180 top
C8  18pF  [C0603]  29.34,30.84 180 top
C9  100nF  [C0603]  26.8,30.35 90 top
C10  26.7,33.86 90 top
C11  35.03,33.86 90 top
C12  100nF  [C0603]  34.92,30.35 90 top
C13  100nF  [C0603]  17.86,7.77 270 top
C14  18pF  [C0603]  19.3,34.16 0 top
C15  19.3,28.07 0 top
C16  10uF  [C0805']  19.15,38.23 0 top
C17  100nF  [C0603]  22.86,32.79 180 top
C18  20pF  [C0603]  45.24,33.35 180 top
C19  20pF  [C0603]  42.24,33.35 0 top
C20  100nF  [C0603]  65.86,22.5 270 top
C21  100nF  [C0603]  41.88,13.13 0 top
C22  43.74,41.35 0 top
C23  54.28,13.36 0 top
C24  100nF  [C0603]  13.23,22.94 270 top
C25  100nF  [C0603]  18.97,20.27 180 top
C26  100nF  [C0603]  11.73,22.94 270 top
C27  100nF  [C0603]  15.01,22.94 270 top
C28  100nF  [C0603]  7.85,31.06 180 top
D10  39.12,44.98 0 top
D11  30.48,44.98 0 top
DIO1  33.02,14.66 180 top
F1  15.93,47.09 180 top
FD1  48.18,1.8 0 top
FD2  6.12,51.36 0 top
FD3  4.11,3.56 0 top
ICSP  65.02,27.94 270 top
IOH  30.23,50.8 180 top
IOL  54.61,50.8 180 top
J1  59.36,43.56 0 top
JP1  12.12,33.35 0 top
JP2  13.61,37.57 270 top
JP3  47.12,44.98 90 top
JP4  52.17,20.57 270 top
JP5  52.17,17.83 270 top
L1  42.52,15.11 0 top
L2  64.97,19.46 0 top
LED1  24.84,9.35 0 top
LED2  28.24,9.35 0 top
LED3  31.65,9.35 0 top
LED4  62.92,37.19 0 top
ON  27.53,4.88 270 top
POWER  36.83,2.54 0 top
Q1  19.3,23.62 180 top
Q2  58.22,29.08 270 top
R1  58.45,14.5 180 top
R2  58.24,25.96 270 top
R3  24.36,4.88 0 top
R4  21.18,40.51 180 top
R5  58.24,33.83 90 top
R6  26.54,9.65 270 top
R7  29.95,9.65 270 top
R8  33.35,9.65 270 top
R9  19.3,30.1 180 top
R10  19.3,32.13 180 top
R11  19.3,26.04 0 top
R12  22.86,24.38 180 top
R13  19.3,36.2 0 top
R14  22.86,30.63 0 top
R15  22.86,34.95 0 top
R16  43.74,38.84 0 top
R17  44.4,30.84 90 top
R18  50.24,14.5 180 top
R19  62.92,33.99 90 top
R20  22.86,20.45 180 top
R21  22.86,21.87 180 top
R22  21.18,41.88 0 top
R23  58.45,13.21 180 top
R24  50.24,13.21 180 top
RN1  58.24,22.56 270 top
RN2  58.24,37.41 270 top
RN3  58.24,19.02 270 top
RST1  20.7,5.41 270 top
RST2  63.58,16.08 0 top
T1  21.59,44.35 180 top
T2  10.21,42.67 0 top
TP  24.59,1.88 0 top
U1  30.86,23.62 180 top
U2  5.77,24.13 90 top
U3  52.07,37.47 270 top
U4  52.07,31.12 270 top
U5  52.07,24.77 270 top
U6  10.69,16.89 0 top
U7  15.75,42.42 270 top
U8  13.41,28.02 0 top
U9  42.24,23.62 90 top
UART_DBG  2.87,28.8 90 top
X1  6.15,49.78 180 top
X2  4.83,7.32 90 top
Y1  30.86,33.58 0 top
Y2  43.74,36.09 0 top

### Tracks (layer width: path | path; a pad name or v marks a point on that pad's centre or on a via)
+3V3  (via drill 0.61)
  Top 0.61: U7.5 16.92,40.51 16.03,39.62 11.74,39.62 10.85,40.51 10.85,41.66 | U7.2 12.24,43.05 10.85,41.66 | 10.85,41.66 T2.1 10.24,42.65 v10.26,42.67 | JP1.1 8.43,34.49 | 8.43,34.49 7.68,34.49 C3.1 7.62,34.17 | v4.52,38.07 6.68,35.92 v8.43,35.92 8.43,34.49 | U2.5 4.46,23.19 v3.35,23.19 | TP.P$1 23.19,1.88 v22.94,1.63
  Bottom 0.61: v10.26,42.67 10.26,45.72 8.89,47.09 6.17,47.09 5.77,46.69 5.77,44.17 6.99,42.95 6.99,42.19 7.82,41.35 7.82,36.53 v8.43,35.92 | POWER.4 35.56,1.75 34.49,0.69 22.73,0.69 | 22.73,0.69 17.6,0.69 16.79,1.5 16.79,7.32 4.27,19.84 4.27,22.28 v3.35,23.19 3.35,34.62 4.52,35.79 v4.52,38.07 | v22.94,1.63 22.94,0.89 22.73,0.69
+5V  (via drill 0.61)
  Top 0.61: T1.2 21.54,44.32 U7.8 16.05,44.32 v15.9,44.48 | 38.1,3.43 POWER.5 38.1,3.89 35.84,6.15 23.88,6.15 23.51,5.78 R3.1 21.16,4.88 19.53,6.5 19.53,11.37 C6.+ 16.07,11.71 v14,11.71 11.53,11.71 10.69,12.55 U6.2 | C1.1 10.34,27.03 v11.3,27.99 | C1.1 C2.1 | C1.1 8.7,26.03 7.75,25.08 U2.3 6.11,25.08 5.79,24.77 5.79,23.19 | v6.25,21.46 5.79,21.92 5.79,23.19 | U2.1 7.06,23.19 5.79,23.19 | v11.56,17.91 10.69,18.77 U6.4
  Bottom 0.61: v15.9,44.48 15.9,45.29 11.18,50.01 6.55,50.01 4.7,48.16 4.7,43.66 5.92,42.44 5.92,41.68 6.76,40.84 6.76,35.23 7.42,34.57 13.44,34.57 JP1.3 14.66,31.34 v11.3,27.99 | ICSP.2 67.18,30.48 67.59,30.07 67.59,12.6 58.75,3.76 38.43,3.76 38.1,3.43 POWER.5 | v14,11.71 14,15.47 v11.56,17.91 9.8,17.91 v6.25,21.46
A0
  Top 0.254: U9.43 42.49,17.15 42.7,16.94 44.88,16.94 45.82,16 45.82,5.79 47.8,3.81 49.73,3.81 50.8,2.74 AD.6
A1
  Top 0.254: U9.44 43,19.36 43,17.53 43.23,17.3 45.06,17.3 46.18,16.18 46.18,5.97 47.98,4.17 51.71,4.17 AD.5
A2
  Top 0.254: U9.45 43.49,17.98 43.82,17.65 45.24,17.65 46.53,16.36 46.53,6.15 48.16,4.52 53.9,4.52 AD.4
A3
  Top 0.254: U9.46 43.99,18.34 44.32,18.01 45.42,18.01 46.89,16.54 46.89,6.32 48.34,4.88 56.08,4.88 AD.3
A4(AIN4)
  Top 0.254: U9.47 44.5,19.36 44.5,18.59 44.73,18.36 45.59,18.36 47.24,16.71 47.24,10.82 A4.1
A4(AIN4/SDA)
  Top 0.254: A4.2 50.9,6.58 52.15,5.33 58.17,5.33 AD.2
A4(SDA)  (via drill 0.25)
  Top 0.254: U9.10 45.32,25.37 v45.09,25.6 41.55,22.07 v41.55,21.9 | IOH.9 21.34,49.53 21.74,49.12 24.26,49.12 24.97,48.41 24.97,44.2 27.76,41.4 37.77,41.4 38.46,40.72 38.46,30.2 v38.79,29.87 | R24.1 51.49,12.81 51.49,11.53 v52.25,10.77 52.38,10.77 A4.3
  Bottom 0.254: v45.09,25.6 44.48,26.21 44.48,28.78 43.38,29.87 v38.79,29.87 | A4.3 53.44,8 53.06,7.62 43.31,7.62 42.7,8.23 42.7,12.34 43.74,13.39 43.74,15.42 41.55,17.6 v41.55,21.9
A5(AIN5)/ICSP4(MOSI_0)
  Top 0.254: U9.1 46.49,19.91 47.96,18.44 47.96,12.37 49.68,10.64 51.28,10.64 52.22,9.7 52.22,8.84 53.39,7.67 57.68,7.67 58.5,8.48 58.5,10.26 58.88,10.64 61.14,10.64 A5.1
  Bottom 0.254: ICSP.4 65.18,26.82 65.18,10.97 63.91,9.7 A5.1
A5(AIN5/SCL)
  Top 0.254: AD.1 59.54,6.5 A5.2
A5(SCL)  (via drill 0.25)
  Top 0.254: U9.11 45.71,25.87 v45.09,26.49 40.69,22.1 v40.69,21.9 | v38.43,28.98 38.1,29.31 38.1,40.54 37.59,41.05 27.58,41.05 24.61,44.02 24.61,48.23 24.08,48.77 20.83,48.77 IOH.10 | A5.3 57,10.06 59.3,12.36 R23.1
  Bottom 0.254: v40.69,21.9 41.2,21.39 41.2,17.42 43.38,15.24 43.38,13.56 42.34,12.52 42.34,8.05 43.13,7.26 56.34,7.26 57,7.93 A5.3 | v45.09,26.49 45.09,29.54 44.2,30.43 38.2,30.43 37.95,30.18 37.95,29.46 v38.43,28.98
AGND  (via drill 0.61)
  Top 0.254: 44.88,23.37 U9.6
  Top 0.61: 44.88,23.37 43.97,23.37 42.6,22 v42.6,21.72 | L2.2 66.04,19.46 61.75,15.16 v61.75,14.58
  Bottom 0.61: v42.6,21.72 42.6,17.35 45.92,14.02 61.19,14.02 v61.75,14.58
  pour Top: 62.48,24.46 69.93,24.46 69.93,17.45 62.48,17.45
AVCC  (via drill 0.61)
  Top 0.406: U9.42 41.99,17.01 42.49,16.51 43.82,16.51 44.02,16.31 L1.2
  Top 0.61: C4.1 C20.1 65.67,23.34 66.6,23.34 67.59,22.35 67.59,18.24 67.11,17.75 65.71,17.75 64.29,16.33 v64.29,11.71 | L1.2 45.29,13.84 v45.29,4.67
  Bottom 0.61: v64.29,11.71 61.34,11.71 60.86,11.23 60.86,7.49 58.04,4.67 v45.29,4.67
CMP
  Top 0.254: U7.3 14.25,41.78 14.88,42.42 19.92,42.42 20.33,42 R22.1 R4.2
D0(RXD1)  (via drill 0.25)
  Top 0.254: U9.39 40.49,20.32 41.1,20.93 42.95,20.93 43.64,21.62 v43.64,21.9
  Bottom 0.254: IOL.1 63.37,50.67 63.37,41.5 62.38,40.51 62.38,16.28 60.66,14.55 46.48,14.55 43.64,17.4 v43.64,21.9
D1(TXD1)  (via drill 0.25)
  Top 0.254: U9.40 40.99,20.29 41.28,20.57 43.59,20.57 44.5,21.49 v44.5,21.9
  Bottom 0.254: IOL.2 62.97,48.79 62.97,41.63 62,40.67 62,16.43 60.48,14.91 46.96,14.91 44.5,17.37 v44.5,21.9
D2  (via drill 0.25)
  Top 0.254: U9.24 39.49,26.96 39.75,26.7 43.56,26.7 v43.89,26.37 | IOL.3 58.42,49.1 57.18,47.85 51.13,47.85 50.27,46.99 50.27,40.16 v51.13,39.29
  Bottom 0.254: v43.89,26.37 43.89,25.22 44.12,24.99 46.69,24.99 47.3,25.6 47.3,27.48 47.9,28.09 49,28.09 49.43,28.52 49.43,32.16 51.16,33.88 51.16,36.78 50.75,37.19 50.75,38.91 v51.13,39.29
D3(PWM1)  (via drill 0.25)
  Top 0.254: U9.36 37.56,20.87 37.39,20.7 37.39,17.81 38.74,16.46 38.74,12.95 39.78,11.91 v43.56,11.91
  Bottom 0.254: IOL.4 55.88,52.43 56.24,52.78 64.03,52.78 65.51,51.31 65.51,41.55 65.18,41.22 63.63,41.22 62.74,40.34 62.74,13.94 62.28,13.49 45.14,13.49 v43.56,11.91
D4  (via drill 0.25)
  Top 0.254: U9.48 45.32,19.37 v45.44,19.25
  Bottom 0.254: IOL.5 53.34,48.95 55.65,46.63 60,46.63 60.68,45.95 60.68,41.63 61.65,40.67 61.65,16.61 60.3,15.27 47.47,15.27 45.42,17.32 45.42,19.23 v45.44,19.25
D5(PWM3)  (via drill 0.25)
  Top 0.254: IOL.6 50.8,48.06 49.91,47.17 49.91,43.21 47.65,40.95 47.65,30.61 v48.16,30.1 | v46.33,29.41 46.49,29.25 U9.12
  Bottom 0.254: v48.16,30.1 47.02,30.1 v46.33,29.41
D6(PWM4)
  Top 0.254: IOL.7 48.26,51.99 47.78,52.48 41,52.48 40.23,51.71 40.23,31.88 42.14,29.97 42.14,29.11 41.73,28.7 40.13,28.7 39.99,28.56 U9.23
D7
  Top 0.254: U9.8 47.18,24.37 47.63,24.82 47.63,27.1 47.24,27.48 47.24,46.3 45.72,47.83 IOL.8
D8
  Top 0.254: U9.9 47.07,24.87 47.27,25.07 47.27,26.92 46.89,27.31 46.89,46.13 45.39,47.63 42.22,47.63 41.66,48.18 IOH.1
D9(PWM5)  (via drill 0.25)
  Top 0.254: U9.25 37.74,26.62 37.74,32.41 36.98,33.17 36.98,33.76 37.39,34.16 37.39,39.68 v37.06,40.01
  Bottom 0.254: v37.06,40.01 34.85,42.22 34.85,46.53 35.38,47.07 37.34,47.07 39.12,48.84 IOH.2
D10(PWM6)  (via drill 0.25)
  Top 0.254: U9.26 37.98,25.86 37.41,25.86 37.24,26.04 37.24,32.36 36.63,32.97 36.63,36.93 v36.8,37.11
  Bottom 0.254: v36.8,37.11 41.66,41.96 D10.3
D10(SS1)  (via drill 0.25)
  Top 0.254: U9.35 39.28,21.37 42.75,24.84 v42.75,25.53 | v41.45,29.26 41.45,30.12 39.88,31.7 39.88,41.43 38.48,42.82 36.78,42.82 36.58,43.03 D10.1
  Bottom 0.254: v41.45,29.26 41.45,26.82 v42.75,25.53
D10(SS1/PWM6)
  Top 0.254: IOH.3 36.58,48.34 39.12,45.8 D10.2
D11(MOSI_1)  (via drill 0.25)
  Top 0.254: U9.34 39.25,21.87 41.73,24.36 v41.73,25.48 | D11.1 27.94,43.1 28.58,42.47 38.3,42.47 39.52,41.25 39.52,31.52 40.69,30.35 v40.69,29.26
  Bottom 0.254: v41.73,25.48 40.69,26.52 v40.69,29.26
D11(MOSI_1/PWM7)
  Top 0.254: D11.2 34.04,48.54 IOH.4
D11(PWM7)  (via drill 0.25)
  Top 0.254: v32.94,39.75 35.66,39.75 36.25,39.17 36.25,32.82 36.88,32.18 36.88,25.55 37.06,25.37 U9.27
  Bottom 0.254: v32.94,39.75 32.94,44.91 D11.3
D12(MISO_1)  (via drill 0.25)
  Top 0.254: U9.33 39.21,22.37 40.87,24.03 v40.87,25.4 | IOH.5 31.52,50.77 31.52,49.35 30.94,48.77 26.21,48.77 25.68,48.23 25.68,44.55 28.12,42.11 38.13,42.11 39.17,41.07 39.17,31.34 39.93,30.58 v39.93,29.26
  Bottom 0.254: v40.87,25.4 39.93,26.34 v39.93,29.26
D13(SCK1)  (via drill 0.25)
  Top 0.254: IOH.6 28.96,49.5 28.58,49.12 26.04,49.12 25.32,48.41 25.32,44.37 27.94,41.76 37.95,41.76 38.81,40.89 38.81,31.17 39.34,30.63 39.34,28.75 38.99,28.4 38.99,26.75 40.11,25.63 40.11,23.8 39.18,22.87 U9.32 37.32,22.87 37.03,22.58 37.03,17.63 38.38,16.28 38.38,12.78 40.11,11.05 v43.56,11.05 | R19.1 64.78,33.14 v64.8,33.12
  Bottom 0.254: v64.8,33.12 64.8,13.64 64.29,13.13 45.64,13.13 v43.56,11.05
DBG_VCC  (via drill 0.51)
  Top 0.406: LED2.A 28.45,8.3 | 24.84,8.43 LED1.A 24.84,8.03 | C11.1 34.15,32.91 33.96,33.1 33.96,36.53 v32.61,37.87 | v51.46,43.21 51.46,41.17 53.22,39.42 U3.14 55.76,39.42 v56.06,39.12 | C9.1 27.29,29.01 29.92,29.01 30.11,28.82 U1.8 | R20.2 R21.2 | U1.44 36.18,24.37 36.2,24.38 | C12.1 36.18,29.5 36.2,29.52
  Top 0.508: 24.84,8.43 20.19,13.08 v20.19,13.72 | C11.1 36.2,31.74 36.2,29.52 36.2,24.38 36.2,17.2 37.54,15.85 v37.54,11.48 40.01,9.02 v43.46,9.02 | 24.84,8.03 25.53,7.34 28.25,7.34 | 28.25,7.34 31.65,7.34 | v33.07,7.57 32.84,7.34 31.65,7.34 | LED3.A 31.65,7.34 | LED2.A 28.25,7.34 | v54,11.74 54.2,11.94 54.2,15.47 | U4.14 55.87,33.07 v55.91,33.1 | v55.91,26.72 v55.9,26.72 U5.14 | v56.06,39.12 56.29,39.34 58.14,39.34 RN2.8 RN2.7 RN2.6 | v22.76,36.78 22.01,36.03 R15.1 23.71,33.25 C17.1 24.74,32.79 | C10.1 26.58,32.79 24.74,32.79 | 24.74,32.79 24.74,31.06 26.3,29.5 C9.1 | R21.2 21.39,21.87 v20.78,21.26 20.52,21.51 17.93,21.51 17.2,22.25 17.2,24.62 | T2.2 9.27,44.53 8.59,45.21 8.59,47.02 8.26,47.35 4.17,47.35 3.89,47.07 3.89,44.04 7.16,40.77 7.16,37.92 8.05,37.03 9.04,37.03 9.91,36.17 14.3,36.17 16.56,33.91 16.56,28.25 17.2,27.61 17.2,24.62 | RN3.3 57.6,18.64 arc-90 RN3.3 | Q1.2 17.2,24.62 | 55.37,18.62 55.37,18.09 54.2,16.92 54.2,15.49 | 55.37,18.62 v55.37,20.57 | 55.37,18.62 arc-90 55.4,18.64 55.42,18.62 RN3.3
  Bottom 0.508: v20.19,13.72 20.19,20.68 v20.78,21.26 | v43.46,9.02 46.74,12.29 53.44,12.29 v54,11.74 | v56.06,39.12 55.91,38.96 v55.91,33.1 v55.91,26.72 55.91,21.11 v55.37,20.57 | v22.76,36.78 23.85,37.87 v32.61,37.87 36.6,37.87 37.97,39.24 37.97,46.56 38.84,47.42 47.96,47.42 48.39,46.99 JP3.1 50.17,43.21 v51.46,43.21 | v37.54,11.48 33.63,7.57 v33.07,7.57
DEBUG_MOD  (via drill 0.25)
  Top 0.254: v49.99,26.72 v49.98,26.72 U5.1 | U4.4 v49.99,31.12 52.71,31.12 v53.54,31.95 | U3.3 51.2,38.12 v51.66,38.58 | U5.4 49.84,24.77 v49.99,24.92 50.22,25.15 52.32,25.15 53.36,24.12 U5.10 | U4.10 53.84,30.47 53.54,30.76 v53.54,31.95 | v53.54,31.95 54.01,32.42 U4.13
  Bottom 0.254: v51.66,38.58 51.11,38.02 51.11,37.36 51.51,36.96 51.51,33.71 49.99,32.18 v49.99,31.12 v49.99,26.72 v49.99,24.92
DEBUG_VCC
  Bottom 0.508: J1.1 54.2,42.37 48.46,42.37 JP3.2
DVCC  (via drill 0.51, 0.61)
  Top 0.254: 41.03,15.1 L1.1 41.49,15.58 U9.41 | C21.1 40.96,13.06
  Top 0.406: 11.14,31.06 U8.16
  Top 0.508: JP1.2 11.14,32.37 U8.16 | C28.1 11.14,31.06 | R18.2 R24.2 49.39,12.61 49.71,12.29 50.52,12.29 50.77,12.04 v50.77,11.35 | v57.53,11.66 57.53,13.14 R23.2
  Top 0.61: C21.1 41.02,13.13 L1.1 | 40.96,13.06 40.36,13.06 v39.85,13.56
  Bottom 0.406: 30.48,2.67 POWER.2
  Bottom 0.508: 57.38,10.9 58.09,10.19 58.09,7.75 56.95,6.6 42.82,6.6 41.5,7.93 41.5,11.91 v39.85,13.56 | v50.77,11.35 51.11,11.68 52.88,11.68 53.67,10.9 57.38,10.9 | v57.53,11.66 57.53,11.05 57.38,10.9
  Bottom 0.61: POWER.2 24.51,8.51 17.55,8.51 15.14,10.92 15.14,20.29 9.8,25.63 9.8,31.04 JP1.2 | v39.85,13.56 39.85,12.04 30.48,2.67
GATE_CMD
  Top 0.254: T1.3 20.27,43.66 15.42,43.66 14.76,44.32 U7.1
GND  (via drill 0.3, 0.41, 0.51, 0.61)
  Top 0.305: U1.41 33.64,22.87 33.17,23.34 33.17,25.93 34.16,26.92 34.52,26.92 34.85,27.25 34.85,27.91 34.06,28.7 34.06,30.01 C7.1
  Top 0.406: v21.72,33.66 22.01,33.36 C17.2 | v18.36,39.5 21.02,39.5 R4.1 | v18.39,27.2 18.45,27.2 C15.1 | U9.17 42.99,30.7 41.39,32.3 C19.1 41.39,34.15 v41.5,34.26 | v48.29,29.16 U4.7 50.24,28.07 v53.62,28.07 | C18.1 45.59,32.86 45.59,27.79 v45.75,27.64 | U3.7 50.08,35.52 v50.01,35.51 | 32.1,29.7 31.61,29.21 U1.5 | 32.1,29.7 C7.1 | C8.2 29.13,30.19 v29.13,29.92 | v32.11,29.72 v32.1,29.71 32.1,29.7 | v44.35,8.33 44.32,12.57 44.35,12.6 | RST2.P$1 59.66,15.88 58.95,15.88 v58.83,16 | RN3.2 57.69,19.43 v56.87,19.43 | U8.15 11.79,30.25 11.63,30.1 7.57,30.1 7,30.67 C28.2 | C23.- 55.78,15.88 v56.52,16.61 | v49.73,11.53 49.43,11.53 48.39,12.57 48.39,18.09 v48.87,18.57 | v18.44,33.3 18.45,33.3 C14.1 | U5.7 51.12,22.82 v52.2,21.74 52.2,24.1 v51.97,24.33 | v45.75,39.7 45.24,40.21 C22.-
  Top 0.508: v48.87,18.57 49.5,19.2 54,19.2 v54.51,18.69
  Top 0.61: RST1.P$2 21.79,0.61 28.73,0.61 29.26,1.14 29.26,4.2 ON.C | POWER.6 POWER.7 43.18,6.43 44.35,7.59 44.35,12.6 44.35,12.78 43.99,13.13 C21.2 | C8.2 28.12,31.2 28.09,31.2 | 28.09,31.2 C9.2 | C7.1 33.6,31.2 C12.2 | RST2.P$1 61.24,16.08 63.47,18.31 L2.1 63.09,19.46 62.56,19.99 62.56,25.91 63.3,26.64 65.05,26.64 ICSP.6 | 28.09,31.2 28.09,31.24 27.71,31.24 v27.71,31.62 | U7.4 14.68,40.51 v14.88,40.72 | C16.1 18.34,38.26 v18.36,39.5 | v10.57,37.39 10.57,37.47 10.01,38.02 8.86,38.02 7.82,39.07 7.82,41.07 4.55,44.35 X1.GND | C13.2 16.45,6.92 13.03,10.34 8.28,10.34 X2.3 | J1.5 59.77,42.29 61.09,40.97 63.12,40.97 J1.9 | v45.29,34.29 45.29,34.15 C18.1 | C22.- 44.2,42.39 v44.2,43.21
  Bottom 0.406: v45.75,27.64 47.27,29.16 v48.29,29.16 | v50.01,35.51 49.71,35.81 49.71,39.78 49.15,40.34 46.38,40.34 v45.75,39.7 | v58.83,16 58.83,17.22 58.32,17.73 57.63,17.73 v56.52,16.61 56.79,16.89 | v44.35,8.33 47.55,11.53 v49.73,11.53 | v56.87,19.43 56.87,16.97 | v51.97,24.33 51.97,25.25 53.62,26.9 v53.62,28.07 | v48.87,18.57 49.5,19.2 51.49,19.2 52.2,19.91 v52.2,21.74
  Bottom 0.508: v56.52,16.61 56.52,16.69 v54.51,18.69
  Bottom 0.61: v10.57,37.39 10.57,38.79 12.29,40.51 14.68,40.51 v14.88,40.72 JP2.2 16.36,37.57 | 18.36,39.22 v18.36,39.5 16.43,37.57 16.36,37.57 | v45.29,34.29 44.2,35.38 v44.2,43.21 45.77,41.63 52.78,41.63 53.49,40.92 55.45,40.92 J1.3 | X2.3 5.18,5.23 X2.1 | v18.44,33.3 18.44,35.48 16.36,37.57
  other vias: 30.86,34.21 34.98,35.97 42.62,14.17 24.13,28.98 10.69,22.05 6.43,32.51 5.87,28.27 23.04,40.49 27.76,47.19 64.92,4.95 8.2,24.13 13.26,20.75 16.03,21.54
  pour Bottom (isolate 0.381): -3.05,54 70.46,54 70.46,-0.28 -3.05,-0.28
  pour Top (isolate 0.381): -3.05,54 70.46,54 70.46,24.77 62.1,24.77 62.1,17.04 70.46,17.04 70.46,-0.28 -3.05,-0.28
ICSP1(MISO_0)  (via drill 0.25)
  Top 0.254: v47.32,21.36 46.5,21.36 U9.2 | ICSP.1 61.67,28.4 61.67,18.47 60.48,17.27 58.24,17.27 v57.96,16.99
  Bottom 0.254: v47.32,21.36 47.88,20.8 47.88,17.37 48.51,16.74 51.44,16.74 52.2,15.98 56.95,15.98 v57.96,16.99
ICSP3(SCK0)  (via drill 0.25)
  Top 0.254: v47.27,20.04 47.96,20.73 47.96,21.64 47.6,22 47.02,22 46.89,21.87 U9.3 | ICSP.3 63.75,27.89 62.03,26.16 62.03,18.29 60.63,16.89 58.73,16.89 v57.96,16.13
  Bottom 0.254: v47.27,20.04 47.27,17.45 48.34,16.38 51.26,16.38 52.02,15.62 57.46,15.62 v57.96,16.13
IN_TDO  (via drill 0.25)
  Top 0.254: 56.58,25.42 v56.59,25.4 55.01,25.4 U5.12 | v56.59,31.78 U4.12 | v56.59,22.23 56.66,22.16 RN1.3
  Bottom 0.254: v56.59,22.23 v56.59,25.4 v56.59,31.78
IN_TMS
  Top 0.254: U5.9 57.33,23.47 RN1.1
LATCH_TDI  (via drill 0.25)
  Top 0.254: RN2.1 56.72,38.61 55.58,37.47 U3.11 53.42,37.47 v52.81,38.07 | U5.2 50.42,26.07 51.11,26.75 v52.43,26.75
  Bottom 0.254: v52.81,38.07 52.58,37.85 52.58,26.9 v52.43,26.75
LATCH_TMS  (via drill 0.25)
  Top 0.254: v51.82,30.38 52.38,29.82 U4.9 | U4.3 51.73,31.77 v51.82,31.67 52.25,31.67 v53.59,33.02 | v53.59,34.7 55.47,34.7 56.24,35.46 56.24,36.63 56.62,37.01 RN2.3
  Bottom 0.254: v53.59,34.7 v53.59,33.02 | v51.82,30.38 v51.82,31.67
MCU_SWDCLK  (via drill 0.25)
  Top 0.254: U9.30 37.01,23.87 37.01,23.88 36.68,23.55 36.68,17.45 38.02,16.1 38.02,12.6 40.41,10.21 v43.56,10.21 | v55.55,11.63 55.02,11.63 54.69,11.96 54.69,16.23 v55.12,16.66
  Bottom 0.254: v43.56,10.21 46.13,12.78 54.33,12.78 v55.55,11.63 | v55.12,16.66 54.79,16.33 52.4,16.33 JP5.1
MCU_SWDIO  (via drill 0.25)
  Top 0.254: U9.31 39.15,23.37 39.52,23.75 v39.52,24.69 | v48.21,27.05 48.01,26.85 48.01,22.12 49.56,20.57 JP4.1
  Bottom 0.254: v39.52,24.69 39.93,24.28 47.04,24.28 48.21,25.45 v48.21,27.05
N$1
  Top 0.254: R3.2 ON.A
N$2
  Top 0.61: LED4.A R19.2
N$3
  Top 0.254: U8.1 10.16,24.12 10.16,23.34 10.59,22.91 12.41,22.91 C24.2
N$4
  Top 0.254: U8.3 12.44,24.58 C24.1
N$5  (via drill 0.25)
  Top 0.254: U8.4 13.13,25.14 v13.13,26.9 | v17.22,20.27 C25.2
  Bottom 0.254: v13.13,26.9 13.13,23.09 15.95,20.27 v17.22,20.27
N$6
  Top 0.254: U8.5 13.74,25.95 14,26.21 16.28,26.21 16.71,25.78 16.71,22.02 17.7,21.03 19.61,21.03 19.82,20.82 C25.1
N$7
  Top 0.254: U7.7 15.37,43.05 14.73,43.69 T2.3
N$8  (1 unrouted)
  Top 0.254: U8.14 12.45,30.92 12.45,30.07 12.01,29.64 3.4,29.64 1.73,31.32 0.46,31.32
N$11
  Top 0.254: U8.2 11.79,24.12 C26.1
N$12
  Top 0.254: C27.1 14.39,24.41 U8.6
N$13
  Top 0.254: R9.2 18.45,30.8 18.36,30.89 17.4,30.89 17.04,31.24 17.04,38.3 17.02,38.33 16.89,38.46 16.71,38.63 9.04,38.63 8.36,39.32 8.36,41.76 7.54,42.57 7.54,43.18 6.15,44.58 X1.D+
N$14
  Top 0.254: Q1.3 19.3,25.19 R11.2
N$15
  Top 0.254: R10.2 18.45,31.36 18.34,31.24 17.63,31.24 17.4,31.47 17.4,38.48 16.89,38.99 9.22,38.99 8.71,39.5 8.71,41.94 7.9,42.75 7.9,43.36 6.95,44.31 X1.D-
N$16
  Top 0.254: R12.2 22.01,24.33 | R21.1 23.71,22.68 R12.2 | R12.2 21.97,24.34 20.25,24.34 Q1.1
N$17
  Top 0.254: R8.2 33.24,8.8 LED3.C
N$19
  Top 0.254: R7.2 29.84,8.8 LED2.C
N$32
  Top 0.254: LED1.C 24.95,10.4 R6.2
N$33  (via drill 0.25)
  Top 0.254: v59.64,18.52 59.53,18.62 RN3.6 | 59.89,28.93 59.64,29.18 59.42,29.18 Q2.3 59.32,27.16 v59.13,26.98 58.22,26.98 | 58.18,26.98 58.22,26.98 | R2.1 58.22,26.81 58.22,26.98
  Bottom 0.254: v59.64,18.52 60.45,19.33 60.45,23.42 58.67,25.2 58.67,26.52 v59.13,26.98
N$40
  Top 0.254: R17.2 44.8,31.75 | R16.2 44.59,37.36 Y2.2 44.39,34.65 C18.2 44.4,33.34 R17.2 | 44.52,31.59 R17.2
N$41  (via drill 0.25)
  Top 0.254: RN3.8 RN3.7 v59.58,19.42 v59.59,19.43 | 58.86,30.97 v58.88,30.99 58.07,30.99 Q2.1
  Bottom 0.254: v58.88,30.99 58.22,30.33 58.22,25.12 60.1,23.24 60.1,19.94 v59.59,19.43
N$42  (1 unrouted)
  Top 0.254: U8.13 13.09,29.8 12.57,29.29 1.5,29.29 0.79,28.58
N$43
  Top 0.254: U9.18 42.49,30.15 40.59,32.06 40.59,41.45 40.82,41.68 42.04,41.68 C22.+
NC/TDI
  Top 0.254: J1.8 60.78,43.71 58.34,43.71 57.94,43.31 57.94,41.28 58.29,40.92 59.54,40.92 60.96,39.5 60.96,22.78 59.53,21.36 RN1.5
NRESET  (via drill 0.25)
  Top 0.254: J1.10 62.97,43.36 58.52,43.36 58.29,43.13 58.29,41.45 58.47,41.28 59.72,41.28 61.32,39.68 61.32,21.82 v61.06,21.56 61.06,18.39 60.6,17.93 57.81,17.93 57.25,17.37 57.25,14.5 R1.2 | R2.2 58.89,25.76 v59.54,25.76
  Bottom 0.254: v61.06,21.56 61.06,24.23 v59.54,25.76
OUT_TDI  (via drill 0.25)
  Top 0.254: U4.6 49.17,29.79 51.51,29.79 v51.82,29.49 | RN1.4 57.36,21.62 53.09,21.62 52.35,20.88 51.99,20.88 51.36,21.51 49.15,21.51 48.39,22.28 48.39,25.3 48.5,25.42 U5.3 49.62,25.42 49.86,25.65 51.38,25.65 v51.79,26.06
  Bottom 0.254: v51.82,29.49 51.79,29.46 v51.79,26.06
OUT_TMS
  Top 0.254: R5.2 56.17,34.68 55.07,33.58 48.51,33.58 48.11,33.99 48.11,35.99 48.28,36.17 U3.6
PIO000  (via drill 0.25)
  Top 0.254: U1.3 32.61,26.74 31.7,25.83 v28.42,25.83 | 20.73,9.12 RST1.P$1 21.46,9.88 v21.49,9.88 | C13.1 17.86,9.3 18.44,9.88 v18.57,9.88 | v24.79,20.42 23.74,20.42 arc-90 R20.1
  Bottom 0.254: v18.57,9.88 v21.49,9.88 21.49,18.9 23.01,20.42 v24.79,20.42 24.79,22.2 v28.42,25.83
PIO001  (via drill 0.25)
  Top 0.254: v24.82,34.95 R15.2 23.71,36.84 27.56,40.69 37.41,40.69 37.74,40.36 37.74,33.68 v37.54,33.48 | U1.4 32.11,28.66 33.07,29.62 v33.43,29.62
  Bottom 0.254: v37.54,33.48 36.42,33.48 33.43,30.48 v33.43,29.62 | v24.82,34.95 22.83,34.95 22.05,35.74 22.05,38.81 17.98,42.88 15.6,42.88 13.59,44.88 13.59,46.38 12.32,47.65 5.92,47.65 5.23,46.96 5.23,43.92 6.45,42.7 6.45,41.94 7.29,41.1 7.29,35.48 7.67,35.1 11.51,35.1 12.34,35.94 JP2.1
PIO003
  Top 0.254: U1.14 25.94,25.87 25.73,26.09 25.73,28.74 R14.2 23.71,30.76 22.67,31.8 21.39,31.8 21.08,32.11 21.08,35.27 R13.2
PIO006
  Top 0.254: U1.22 25.19,21.87 23.71,23.36 R12.1
PIO008  (via drill 0.25)
  Top 0.254: U4.11 v54.18,31.12 | U1.27 29.11,21.05 v28.5,21.67 | v54.18,34.14 v49.56,34.14 | v54.18,35.51 U3.8
  Bottom 0.254: v54.18,31.12 v54.18,34.14 v54.18,35.51 | v28.5,21.67 28.52,21.69 29.57,21.69 30.68,22.81 30.68,24.77 32.72,26.8 34.37,26.8 36.88,29.31 36.88,30.71 37.67,31.5 46.05,31.5 48.67,34.11 49.56,34.11 v49.56,34.14
PIO009  (via drill 0.25)
  Top 0.254: v29.72,20.78 29.61,20.67 U1.28 | U4.5 50.49,30.47 v50.6,30.35 | U5.5 50.12,24.12 v50.17,24.16
  Bottom 0.254: v29.72,20.78 31.39,22.45 31.39,23.55 31.78,23.93 49.94,23.93 v50.17,24.16 50.6,24.59 v50.6,30.35
PIO106  (via drill 0.25)
  Top 0.254: v33.81,25.35 34.94,25.35 U1.46 | U5.11 53.49,24.77 53.04,25.22 53.04,27.18 52.73,27.48 v49.25,27.48
  Bottom 0.254: v33.81,25.35 33.91,25.25 39.9,25.25 40.51,24.64 46.86,24.64 47.65,25.43 47.65,27.31 48.08,27.74 49,27.74 v49.25,27.48
PIO200  (via drill 0.25)
  Top 0.254: U1.2 33.11,26.71 31.88,25.48 28.96,25.48 v28.42,24.94 | v26.54,16.41 R6.1
  Bottom 0.254: v28.42,24.94 26.54,23.06 v26.54,16.41
PIO201  (via drill 0.25)
  Top 0.254: U1.13 v26.76,26.99 v26.77,27 | R7.1 29.95,11.33 27.74,13.54 v27.74,18.11
  Bottom 0.254: v27.74,18.11 27.74,22.4 28.98,23.65 28.98,26.39 28.37,27 v26.77,27
PIO202
  Top 0.254: R8.1 33.35,11.43 32.94,11.84 30.35,11.84 28.61,13.58 U1.26
PIO203  (via drill 0.25)
  Top 0.254: U1.38 34.08,21.37 32.74,22.71 32.74,23.7 v31.85,24.59 | v51.21,40.26 52.7,38.77 U3.13
  Bottom 0.254: v51.21,40.26 50.39,39.45 50.39,37.01 50.8,36.6 50.8,34.06 47.52,30.79 38.02,30.79 37.59,30.35 37.59,28.96 34.72,26.09 33.02,26.09 31.85,24.92 v31.85,24.59
PIO204  (via drill 0.25)
  Top 0.254: v25.55,23.98 25.66,23.87 U1.18 | U4.1 51.47,33.07 v52.02,32.51
  Bottom 0.254: v25.55,23.98 25.55,27.33 32.26,34.04 37.8,34.04 38.56,33.27 45.21,33.27 47.09,35.15 47.09,36.75 44.83,39.01 44.83,40.23 45.42,40.82 51.87,40.82 52.22,40.46 52.22,32.72 v52.02,32.51
PIO205  (via drill 0.25)
  Top 0.254: U3.4 v48.36,37.47 | U1.21 27.83,22.37 28.47,23.01 v29.59,23.01
  Bottom 0.254: v29.59,23.01 30.33,23.75 30.33,24.94 33.5,28.12 34.62,28.12 36.17,29.67 36.17,31.06 37.31,32.21 45.69,32.21 48.16,34.67 48.16,37.26 v48.36,37.47
PIO206  (via drill 0.25)
  Top 0.254: v49.02,34.87 51.05,34.87 53,36.82 U3.10 | 33.61,27.97 U1.1 33.77,27.56 v34.11,27.56
  Bottom 0.254: v34.11,27.56 34.6,27.56 36.53,29.49 36.53,30.89 37.49,31.85 45.87,31.85 48.9,34.87 v49.02,34.87
PIO207  (via drill 0.25)
  Top 0.254: U1.11 28.61,26.81 29.03,26.39 v30.35,26.39 | v48.36,38.76 v48.37,38.77 U3.2
  Bottom 0.254: v30.35,26.39 31.24,26.39 33.33,28.47 34.44,28.47 35.81,29.85 35.81,31.24 37.14,32.56 45.52,32.56 47.8,34.85 47.8,38.2 v48.36,38.76
PIO208  (via drill 0.25)
  Top 0.254: v28.42,23.98 27.86,24.59 27.86,27.48 U1.12 | RN3.1 56.58,21.26 54.74,21.26 v54.53,21.06
  Bottom 0.254: v28.42,23.98 26.9,22.4 26.9,18.03 27.51,17.42 29.62,17.42 34.7,22.5 53.09,22.5 v54.53,21.06
PIO209  (via drill 0.25)
  Top 0.254: v53.95,38.1 54.98,38.1 U3.12 | U1.24 27.73,20.87 27.89,21.03 27.89,21.9 28.22,22.23 31.12,22.23 v31.65,21.69
  Bottom 0.254: v53.95,38.1 52.93,37.08 52.93,31.32 54.43,29.82 54.43,25.3 52.35,23.22 33.17,23.22 v31.65,21.69
PIO210  (via drill 0.25)
  Top 0.254: 28.12,19.5 U1.25 28.11,20.39 v28.5,20.78 | U4.2 48.37,32.42 v48.23,32.41
  Bottom 0.254: v28.5,20.78 29.06,21.34 29.74,21.34 31.04,22.63 31.04,24.61 32.87,26.44 34.54,26.44 37.24,29.13 37.24,30.53 37.85,31.14 47.35,31.14 48.23,32.03 v48.23,32.41
PIO211  (via drill 0.25)
  Top 0.254: v31.12,20.85 U1.31 | RN1.2 56.41,22.96 55.63,22.17 v55.07,22.17
  Bottom 0.254: v55.07,22.17 54.38,22.86 33.96,22.86 31.95,20.85 v31.12,20.85
PIO300  (via drill 0.25)
  Top 0.254: U3.1 48.6,39.42 v48.36,39.65 | v29.54,24.92 29.54,24.71 33.61,20.64 U1.36
  Bottom 0.254: v48.36,39.65 47.45,38.74 47.45,35 45.36,32.92 36.96,32.92 35.46,31.42 35.46,30.02 34.26,28.83 33.15,28.83 31.29,26.98 30.1,26.98 29.54,26.42 v29.54,24.92
PIO301  (via drill 0.25)
  Top 0.254: U1.37 34.07,20.87 32.11,22.83 v32.11,23.27 | v53.82,26.06 U5.13
  Bottom 0.254: v32.11,23.27 32.41,23.57 52.17,23.57 53.82,25.22 v53.82,26.06
PWRIN  (via drill 0.41)
  Top 0.406: v22.23,6.78 33.86,6.78 34.39,7.32 34.39,11.68 33.38,12.7 31.78,12.7 30.82,13.66 DIO1.A | v18.69,5.77 14.05,5.77 13.54,5.77 12.65,5.77 X2.2
  Bottom 0.406: v22.23,6.78 21.21,5.77 v18.69,5.77
RESET  (via drill 0.25)
  Top 0.254: U9.4 45.51,22.37 45.36,22.23 45.36,20.47 46.46,19.38 v46.46,18.97 47.6,17.83 47.6,12.19 49.66,10.13 v49.66,5.54 | C23.+ 52.78,11.3 53.34,10.74 54.41,10.74 55.14,10.01 55.14,9.17 55.73,8.59 57.63,8.59 58.06,9.02 58.06,10.54 59.61,12.09 60.15,12.09 60.78,12.73 60.78,13.69 | v63.37,13.69 63.37,13.46 | v63.37,13.69 63.37,11.15 64.08,10.44 66.55,10.44 67.28,11.18 RST2.P$2 | C23.+ 52.78,15.14 52.1,15.82 v51,15.82 | C23.+ 51.64,14.5 R18.1 | 60.78,13.69 59.97,14.5 R1.1 | v63.37,13.69 60.78,13.69
  Bottom 0.254: POWER.3 33.02,4.22 34.34,5.54 v49.66,5.54 | ICSP.5 63.37,25.02 v63.37,13.69 | v51,15.82 47.93,15.82 46.46,17.3 v46.46,18.97
RXD  (via drill 0.25)
  Top 0.254: U8.12 13.74,31.49 13.97,31.72 15.9,31.72 16.08,31.55 16.08,28.22 15.34,27.48 12.42,27.48 9.63,24.69 9.63,22.91 8.46,21.74 8.46,18.36 9.75,17.07 15.93,17.07 16.97,16.03 25.32,16.03 v25.53,15.82 | U9.37 39.02,18.9 v38.99,18.9
  Bottom 0.254: v25.53,15.82 25.96,15.39 35.76,15.39 38.99,18.62 v38.99,18.9
SPI_MISO  (via drill 0.25)
  Top 0.254: v53.49,36.17 arc90 v53.5,36.17 U3.9 | U5.8 54.02,22.82 53.65,23.19 v53.65,23.47
  Bottom 0.254: v53.49,36.17 54.58,36.17 54.79,35.97 54.79,24.61 v53.65,23.47
SPI_MOSI  (via drill 0.25)
  Top 0.254: v51.21,28.85 53.67,28.85 53.98,29.17 U4.8 55.63,29.17 55.98,29.52 55.98,30.81 56.34,31.17 v57.2,31.17 | v56.9,37.82 RN2.2 | v51.66,37.64 50.84,36.82 U3.5 | U5.6 50.8,23.47 51.08,23.75 v51.08,24.21
  Bottom 0.254: v57.2,31.17 57.2,37.52 v56.9,37.82 | v51.66,37.64 51.87,37.44 51.87,33.53 51.21,32.87 v51.21,28.85 51.21,24.33 v51.08,24.21
SWDCLK/TCLK  (via drill 0.25)
  Top 0.254: J1.4 55.58,43.59 53.04,43.59 52.68,43.23 52.68,41.12 53.59,40.21 59.18,40.21 60.25,39.14 60.25,23.67 v59.54,22.96 59.56,22.96 RN1.7
  Bottom 0.254: v59.54,22.96 59.28,22.96 55.83,19.51 53.8,19.51 53.44,19.15 JP5.2
SWDIO/TMS  (via drill 0.25)
  Top 0.254: J1.2 53.21,44.83 52.32,43.94 52.32,40.95 53.42,39.85 59,39.85 59.89,38.96 59.89,33.5 59.37,32.98 R5.1 v58.24,31.9 | v57.23,24.61 57.53,24.31 58.14,24.31 58.69,23.76 RN1.8
  Bottom 0.254: v58.24,31.9 57.81,31.47 57.81,25.2 v57.23,24.61 57.23,21.44 55.68,19.89 54.13,19.89 JP4.2
SWO/TDO
  Top 0.254: RN1.6 59.8,22.16 60.6,22.96 60.6,39.32 59.36,40.56 56.24,40.56 55.55,41.25 55.55,42.98 56.13,43.56 57.66,43.56 58.93,44.83 J1.6
TXD  (via drill 0.25)
  Top 0.254: U9.38 39.99,18.2 v39.98,18.19 | U8.11 14.39,28.69 13.59,27.89 12.29,27.89 9.27,24.87 9.27,23.09 8.1,21.92 8.1,18.19 9.58,16.71 15.75,16.71 16.79,15.67 24.46,15.67 v25.78,14.35
  Bottom 0.254: v39.98,18.19 36.14,14.35 v25.78,14.35
USB_DM
  Top 0.254: U1.19 25.19,23.37 24.94,23.62 24.94,27.66 24.51,28.09 21.44,28.09 21.29,28.25 21.29,30.61 21.01,30.89 20.42,30.89 20.15,31.15 R10.1 C14.2
USB_DP
  Top 0.254: U1.20 26.76,22.89 25.15,22.89 24.59,23.44 24.59,27.48 24.33,27.74 21.26,27.74 20.93,28.07 | R9.1 20.78,30.1 20.93,29.95 20.93,28.07 | 20.93,28.07 C15.2 20.15,27.74 R11.1
USBVCC  (via drill 0.41)
  Top 0.406: 18.64,41.78 U7.6 18.25,41.68 v16.82,41.68 | R13.1 20,37.74 C16.2 v21.31,38.23 22.66,38.23 24.71,40.28 24.71,43 22.35,45.36 T1.1 19.6,45.36 F1.1
  Bottom 0.406: v16.82,41.68 18.03,41.68 21.31,38.41 v21.31,38.23
VIN  (via drill 0.41)
  Top 0.406: v25.6,13.26 24.32,13.26 C5.+ 22.34,15.24 16.59,15.24 15.55,16.28 12.85,16.28 | v6.32,19.33 9.37,16.28 12.85,16.28 | DIO1.C arc90 35.02,14.45 v35.02,13.03 | POWER.8 45.72,1.3 45.16,0.74 37.11,0.74 36.83,1.02 36.83,3.81 35.36,5.28 v31.24,5.28 | R22.2 22.16,42.01 v22.96,42.01 | U6.3 13.01,16.13 12.85,16.28
  Bottom 0.406: v22.96,42.01 20.09,42.01 11.46,50.65 4.09,50.65 2.69,49.25 2.69,44.78 5.31,42.16 5.31,41.4 6.15,40.56 6.15,36.14 4.27,34.26 4.27,24.44 5.31,23.39 5.31,20.35 v6.32,19.33 | v25.6,13.26 34.79,13.26 v35.02,13.03 31.24,9.26 v31.24,5.28
XTAL1
  Top 0.254: U9.16 43.49,32.95 C19.2 43.09,34.65 Y2.1 42.89,37.37 R16.1
XTAL2
  Top 0.254: R17.1 43.99,29.58 U9.15
XTALIN
  Top 0.254: U1.6 31.11,30.41 C7.2 31.54,32.16 Y1.2
XTALOUT
  Top 0.254: U1.7 30.61,30.84 C8.1 30.19,32.16 Y1.1
XUSB  (via drill 0.61)
  Top 0.61: F1.2 13.56,46.89 v12.47,45.8 | v9.91,39.78 9.4,40.28 9.4,42.04 8.43,43 8.43,43.61 7.75,44.3 X1.VBUS
  Bottom 0.61: v9.91,39.78 12.47,42.34 v12.47,45.8

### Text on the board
tPlace: TX | RX | + | + | + | + | + | + | +
tNames: 11 | 10 | ~9 | 8 | 7 | ~6 | ~5 | 4 | ~3 | 2 | 1 | 0 | SCL | SDA | GND | ^13 | ^12 | DIGITAL | (PWM~ SPI^) | AREF | 2 | ^1 | ~3 | ^1 | ~3 | 1 | (JTAG/SW) | 1 | 3 | 3 | 1 | 3 | 1 | ANALOG IN | IOREF | RESET | 3.3V | 5V | GND | GND | Vin | A0 | A1 | A2 | A3 | A4 | A5 | +3V3
Measures: 68.52 | mm | mm
214bmp: D:/SmartProjects/Snc/a4_bn_logo2.bmp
